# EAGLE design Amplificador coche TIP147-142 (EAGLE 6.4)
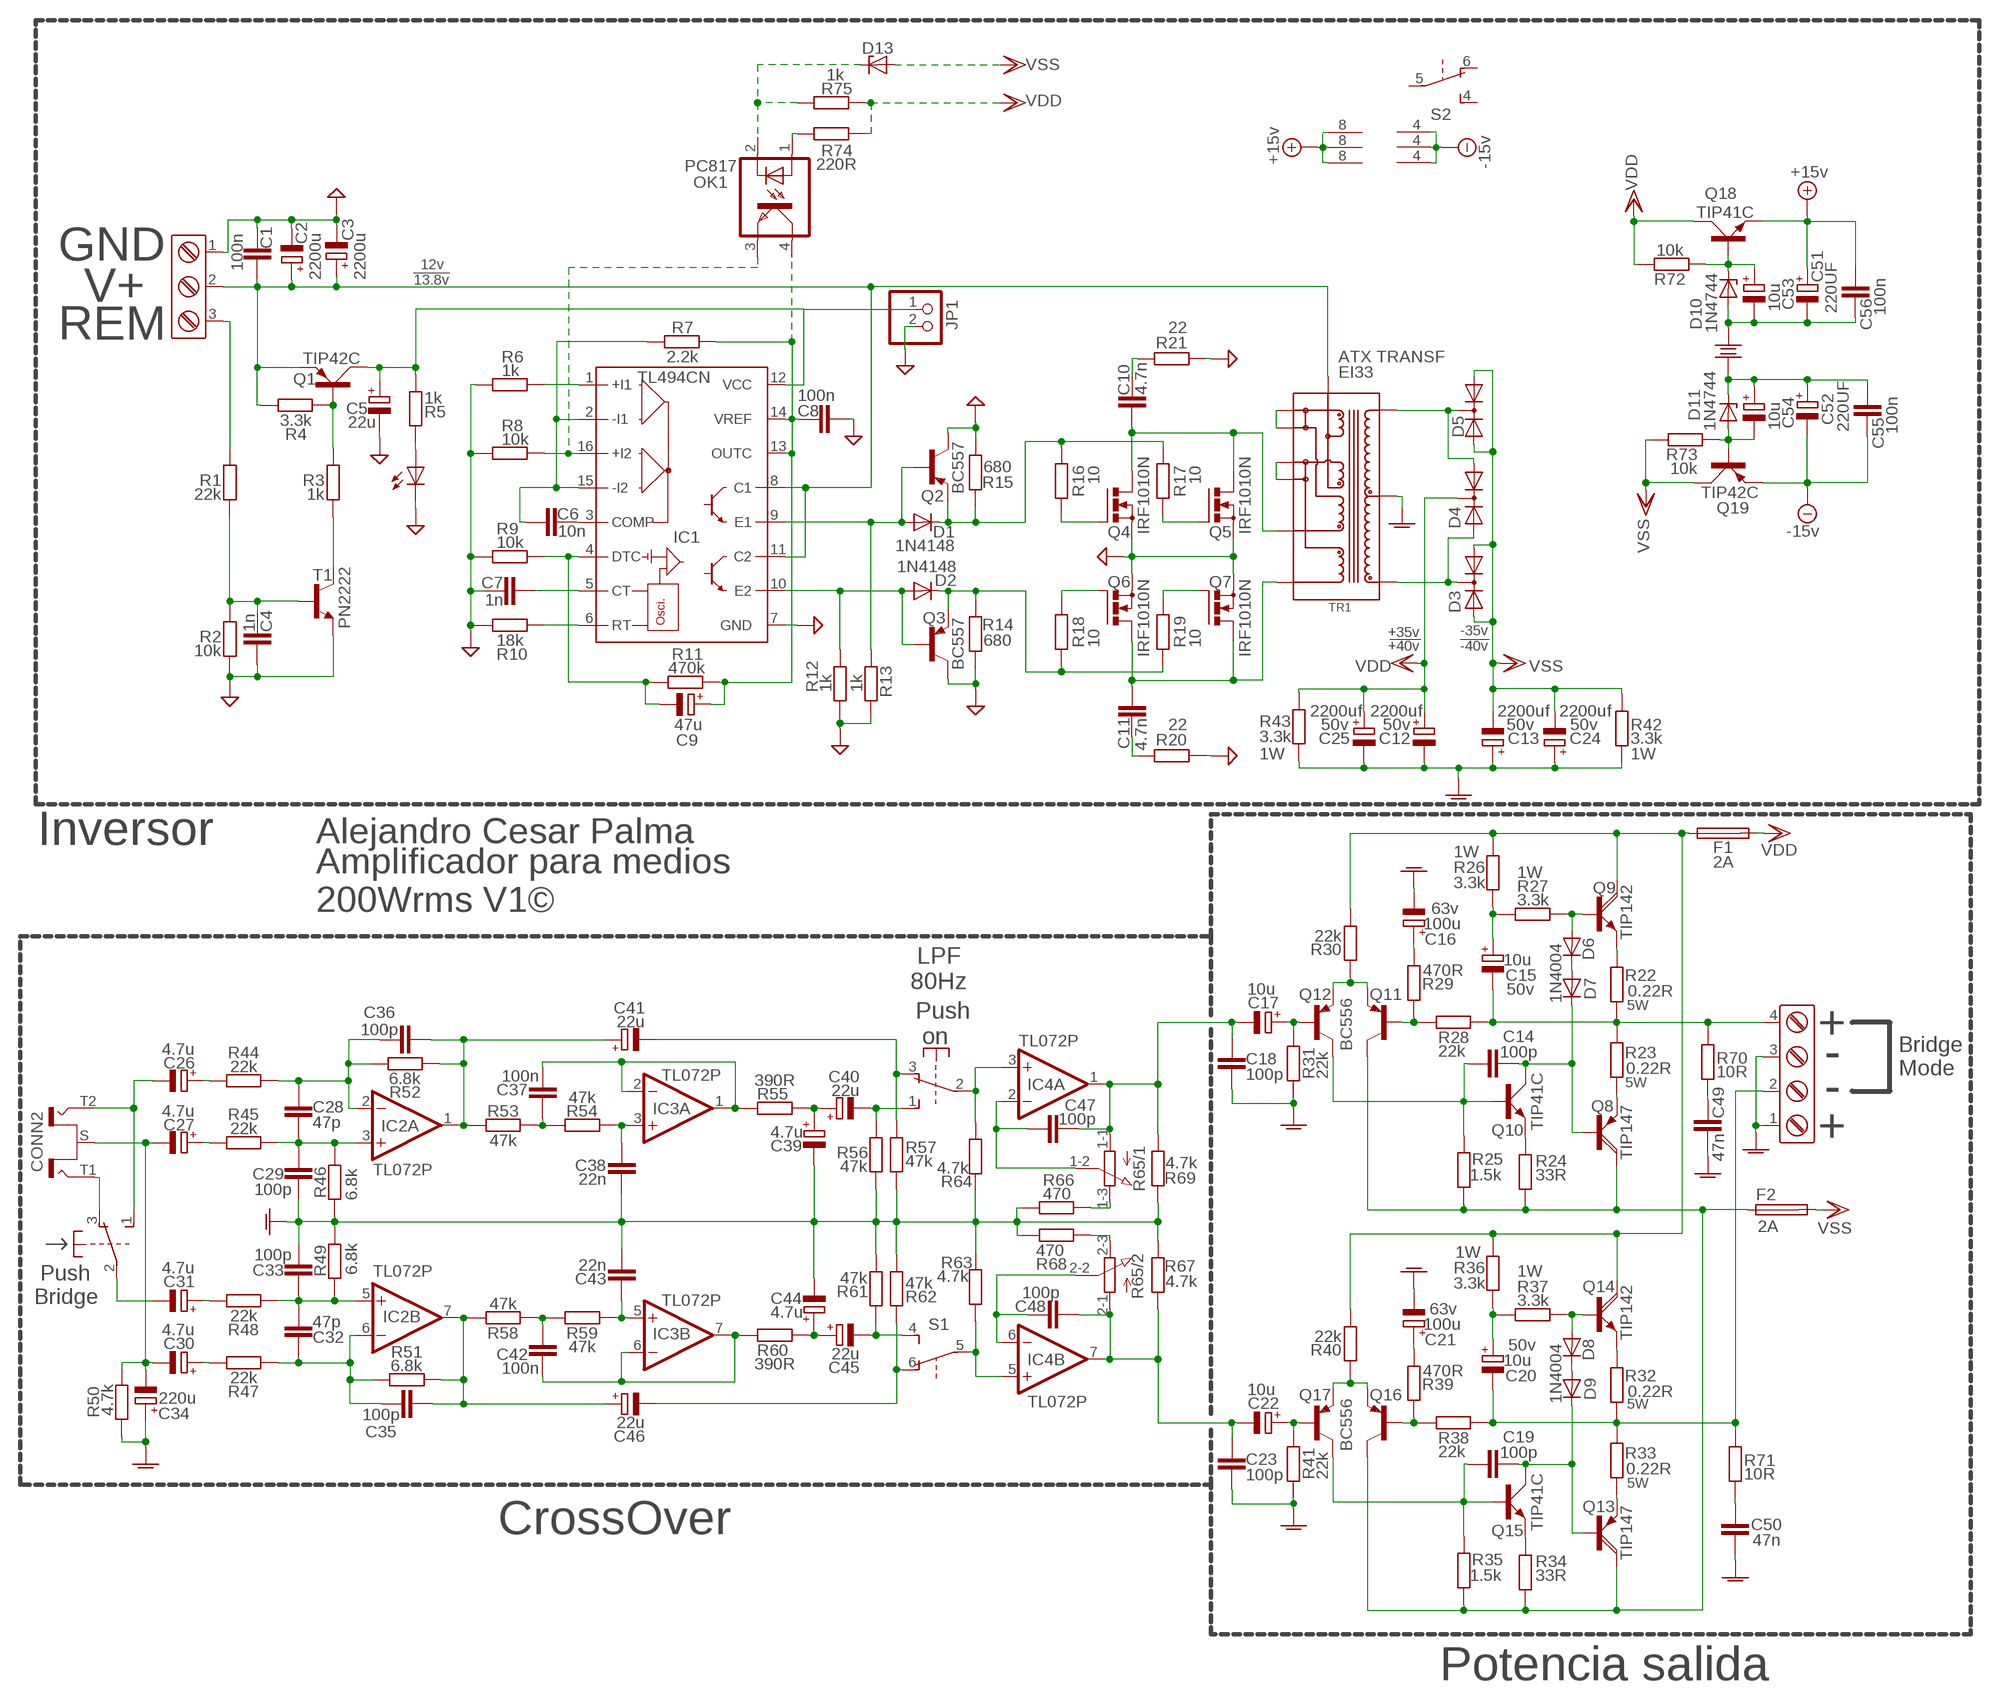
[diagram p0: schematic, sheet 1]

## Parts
C1  100n  C-EU050-024X044  [C050-024X044]
C2  2200u  CPOL-EUE5-13  [E5-13]
C3  2200u  CPOL-EUE5-13  [E5-13]
C4  1n  C-EU050-024X044  [C050-024X044]
C5  22u  CPOL-EUE2.5-5  [E2,5-5]
C6  10n  C-EU050-024X044  [C050-024X044]
C7  1n  C-EU050-024X044  [C050-024X044]
C8  100n  C-EU050-024X044  [C050-024X044]
C9  47u  CPOL-EUE2.5-5  [E2,5-5]
C10  4.7n  C-EU050-024X044  [C050-024X044]
C11  4.7n  C-EU050-024X044  [C050-024X044]
C12  2200uf  CPOL-EUE7.5-18  [E7,5-18]
C13  2200uf  CPOL-EUE7.5-18  [E7,5-18]
C14  100p  C-EU050-024X044  [C050-024X044]
C15  10u  CPOL-EUE2.5-5  [E2,5-5]
C16  100u  CPOL-EUE3.5-8  [E3,5-8]
C17  10u  CPOL-EUE2.5-5  [E2,5-5]
C18  100p  C-EU050-024X044  [C050-024X044]
C19  100p  C-EU050-024X044  [C050-024X044]
C20  10u  CPOL-EUE2.5-5  [E2,5-5]
C21  100u  CPOL-EUE3.5-8  [E3,5-8]
C22  10u  CPOL-EUE2.5-5  [E2,5-5]
C23  100p  C-EU050-024X044  [C050-024X044]
C24  2200uf  CPOL-EUE7.5-18  [E7,5-18]
C25  2200uf  CPOL-EUE7.5-18  [E7,5-18]
C26  4.7u  CPOL-EUE2.5-5  [E2,5-5]
C27  4.7u  CPOL-EUE2.5-5  [E2,5-5]
C28  47p  C-EU050-024X044  [C050-024X044]
C29  100p  C-EU050-024X044  [C050-024X044]
C30  4.7u  CPOL-EUE2.5-5  [E2,5-5]
C31  4.7u  CPOL-EUE2.5-5  [E2,5-5]
C32  47p  C-EU050-024X044  [C050-024X044]
C33  100p  C-EU050-024X044  [C050-024X044]
C34  220u  CPOL-EUE3.5-8  [E3,5-8]
C35  100p  C-EU050-024X044  [C050-024X044]
C36  100p  C-EU050-024X044  [C050-024X044]
C37  100n  C-EU050-024X044  [C050-024X044]
C38  22n  C-EU050-024X044  [C050-024X044]
C39  4.7u  CPOL-EUE2.5-5  [E2,5-5]
C40  22u  CPOL-EUE2.5-5  [E2,5-5]
C41  22u  CPOL-EUE2.5-5  [E2,5-5]
C42  100n  C-EU050-024X044  [C050-024X044]
C43  22n  C-EU050-024X044  [C050-024X044]
C44  4.7u  CPOL-EUE2.5-5  [E2,5-5]
C45  22u  CPOL-EUE2.5-5  [E2,5-5]
C46  22u  CPOL-EUE2.5-5  [E2,5-5]
C47  100p  C-EU050-024X044  [C050-024X044]
C48  100p  C-EU050-024X044  [C050-024X044]
C49  47n  C-EU050-024X044  [C050-024X044]
C50  47n  C-EU050-024X044  [C050-024X044]
C51  220UF  CPOL-EUE5-10.5  [E5-10,5]
C52  220UF  CPOL-EUE5-10.5  [E5-10,5]
C53  10u  CPOL-EUE2.5-5  [E2,5-5]
C54  10u  CPOL-EUE2.5-5  [E2,5-5]
C55  100n  C-EU050-024X044  [C050-024X044]
C56  100n  C-EU050-024X044  [C050-024X044]
CON1  CONECTOR_DEGSON_4_PIN  [CONN_DEGSON_4_PIN]
CONN1  CONECTOR_DEGSON_3_PIN  [CONN_DEGSON_3_PIN]
CONN2  RCA-2-VERT-V2  [RCA-2-VERT_V2]
D1  1N4148  1N4148DO35-7  [DO35-7]
D2  1N4148  1N4148DO35-7  [DO35-7]
D3  FEP16AT  [TO220ABS]
D4  FEP16AT  [TO220ABS]
D5  FEP16AT  [TO220ABS]
D6  1N4004  [DO41-10]
D7  1N4004  [DO41-10]
D8  1N4004  [DO41-10]
D9  1N4004  [DO41-10]
D10  1N4744  ZENER-DIODEDO34-7  [DO34Z7]
D11  1N4744  ZENER-DIODEDO34-7  [DO34Z7]
D13  ZENER-DIODEDO34-7  [DO34Z7]
F1  FUSESHK20L  [SHK20L]
F2  FUSESHK20L  [SHK20L]
IC1  TL494CN  [DIL16]
IC2  TL072P  [DIL08]
IC3  TL072P  [DIL08]
IC4  TL072P  [DIL08]
JP1  PINHD-1X2  [1X02]
LED1  LED3MM  [LED3MM]
OK1  PC817  [DIL04]
Q1  TIP42C  [TO220AV]
Q2  BC557  [TO92-EBC]
Q3  BC557  [TO92-EBC]
Q4  IRF1010N  BUZ11BV  [TO220BV]
Q5  IRF1010N  BUZ11BV  [TO220BV]
Q6  IRF1010N  BUZ11BV  [TO220BV]
Q7  IRF1010N  BUZ11BV  [TO220BV]
Q8  TIP147  [TO247BV]
Q9  TIP142  [TO247BV]
Q10  TIP41C  [TO220AV]
Q11  BC556  [TO92-EBC]
Q12  BC556  [TO92-EBC]
Q13  TIP147  [TO247BV]
Q14  TIP142  [TO247BV]
Q15  TIP41C  [TO220AV]
Q16  BC556  [TO92-EBC]
Q17  BC556  [TO92-EBC]
Q18  TIP41C  [TO220AV]
Q19  TIP42C  [TO220AV]
R1  22k  R-EU_0207/7  [0207/7]
R2  10k  R-EU_0207/7  [0207/7]
R3  1k  R-EU_0207/7  [0207/7]
R4  3.3k  R-EU_0207/7  [0207/7]
R5  1k  R-EU_0207/7  [0207/7]
R6  1k  R-EU_0207/7  [0207/7]
R7  2.2k  R-EU_0207/7  [0207/7]
R8  10k  R-EU_0207/7  [0207/7]
R9  10k  R-EU_0207/7  [0207/7]
R10  18k  R-EU_0207/7  [0207/7]
R11  470k  R-EU_0207/7  [0207/7]
R12  1k  R-EU_0207/7  [0207/7]
R13  1k  R-EU_0207/7  [0207/7]
R14  680  R-EU_0207/7  [0207/7]
R15  680  R-EU_0207/7  [0207/7]
R16  10  R-EU_0207/7  [0207/7]
R17  10  R-EU_0207/7  [0207/7]
R18  10  R-EU_0207/7  [0207/7]
R19  10  R-EU_0207/7  [0207/7]
R20  22  R-EU_0207/7  [0207/7]
R21  22  R-EU_0207/7  [0207/7]
R22  0.22R  R-EU_VTA53  [VTA53]
R23  0.22R  R-EU_VTA53  [VTA53]
R24  33R  R-EU_0207/7  [0207/7]
R25  1.5k  R-EU_0207/7  [0207/7]
R26  3.3k  R-EU_0411/12  [0411/12]
R27  3.3k  R-EU_0411/12  [0411/12]
R28  22k  R-EU_0207/7  [0207/7]
R29  470R  R-EU_0207/7  [0207/7]
R30  22k  R-EU_0207/7  [0207/7]
R31  22k  R-EU_0207/7  [0207/7]
R32  0.22R  R-EU_VTA53  [VTA53]
R33  0.22R  R-EU_VTA53  [VTA53]
R34  33R  R-EU_0207/7  [0207/7]
R35  1.5k  R-EU_0207/7  [0207/7]
R36  3.3k  R-EU_0411/12  [0411/12]
R37  3.3k  R-EU_0411/12  [0411/12]
R38  22k  R-EU_0207/7  [0207/7]
R39  470R  R-EU_0207/7  [0207/7]
R40  22k  R-EU_0207/7  [0207/7]
R41  22k  R-EU_0207/7  [0207/7]
R42  3.3k  R-EU_0411/12  [0411/12]
R43  3.3k  R-EU_0411/12  [0411/12]
R44  22k  R-EU_0207/7  [0207/7]
R45  22k  R-EU_0207/7  [0207/7]
R46  6.8k  R-EU_0207/7  [0207/7]
R47  22k  R-EU_0207/7  [0207/7]
R48  22k  R-EU_0207/7  [0207/7]
R49  6.8k  R-EU_0207/7  [0207/7]
R50  4.7k  R-EU_0207/7  [0207/7]
R51  6.8k  R-EU_0207/7  [0207/7]
R52  6.8k  R-EU_0207/7  [0207/7]
R53  47k  R-EU_0207/7  [0207/7]
R54  47k  R-EU_0207/7  [0207/7]
R55  390R  R-EU_0207/7  [0207/7]
R56  47k  R-EU_0207/7  [0207/7]
R57  47k  R-EU_0207/7  [0207/7]
R58  47k  R-EU_0207/7  [0207/7]
R59  47k  R-EU_0207/7  [0207/7]
R60  390R  R-EU_0207/7  [0207/7]
R61  47k  R-EU_0207/7  [0207/7]
R62  47k  R-EU_0207/7  [0207/7]
R63  4.7k  R-EU_0207/7  [0207/7]
R64  4.7k  R-EU_0207/7  [0207/7]
R65  3RP/1610G  [3RP/1610G]
R66  470  R-EU_0207/7  [0207/7]
R67  4.7k  R-EU_0207/7  [0207/7]
R68  470  R-EU_0207/7  [0207/7]
R69  4.7k  R-EU_0207/7  [0207/7]
R70  10R  R-EU_0411/12  [0411/12]
R71  10R  R-EU_0411/12  [0411/12]
R72  10k  R-EU_0207/7  [0207/7]
R73  10k  R-EU_0207/7  [0207/7]
R74  220R  R-EU_0207/7  [0207/7]
R75  1k  R-EU_0207/7  [0207/7]
S1  9077-2  [9077-2]
S2  9077-2  [9077-2]
T1  PN2222  2N2222-NPN-TO92-EBC  [TO92-EBC]
TR1  ATX1  [ATX/300W]

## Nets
+14V: C51.+ C56.2 IC2.8(P:V+) IC3.8(P:V+) IC4.8(P:V+) Q18.E ; supply symbol labelled +15v
-14V: C52.- C55.1 IC2.4(P:V-) IC3.4(P:V-) IC4.4(P:V-) Q19.E ; supply symbol labelled -15v
GND: C1.1 C2.- C3.- C4.2 C5.- C7.1 C8.2 CONN1.1 IC1.7(GND) JP1.2 LED1.K(C) Q2.C Q3.C Q4.S Q5.S Q6.S Q7.S R2.1 R6.2 R8.2 R9.2 R10.2 R12.2 R13.2 R14.2 R15.2 R20.2 R21.2 T1.E
GNDA: C12.- C13.+ C16.- C18.1 C21.- C23.1 C24.+ C25.- C29.1 C33.1 C34.+ C38.2 C39.- C43.2 C44.- C49.1 C50.1 C51.- C52.+ C53.- C54.+ C55.2 C56.1 CON1.1 CON1.3 D10.A D11.C R31.1 R41.1 R42.2 R43.2 R46.1 R49.1 R50.2 R56.2 R57.2 R61.2 R62.2 R63.1 R64.1 R66.2 R67.1 R68.2 R69.1 TR1.9
N$1: C1.2 C2.+ C3.+ CONN1.2 IC1.8(C1) IC1.11(C2) Q1.E R4.2 TR1.7
N$2: C26.+ R44.1
N$3: CONN1.3 R1.2
N$4: C4.1 R1.1 R2.2 T1.B
N$5: R3.1 T1.C
N$6: Q1.B R3.2 R4.1
N$7: C5.+ IC1.12(VCC) JP1.1 Q1.C R5.1
N$8: LED1.A R5.2
N$9: OK1.1(A) R74.1
N$10: C6.2 IC1.3(COMP)
N$11: C6.1 IC1.2(-I1) IC1.15(-I2) R7.2
N$12: C8.1 C9.+ IC1.13(OUTC) IC1.14(VREF) OK1.4(COL) R7.1 R11.1
N$13: IC1.16(+I2) OK1.3(EMIT) R8.1
N$14: Q4.G R16.1
N$15: C9.- IC1.4(DTC) R9.1 R11.2
N$16: C7.2 IC1.5(CT)
N$17: IC1.6(RT) R10.1
N$18: Q5.G R17.1
N$19: C11.2 R20.1
N$20: D2.A IC1.10(E2) Q3.B R12.1
N$21: D1.A IC1.9(E1) Q2.B R13.1
N$22: D1.C Q2.E R15.1 R16.2 R17.2
N$23: Q6.G R18.1
N$24: D2.C Q3.E R14.1 R18.2 R19.2
N$25: Q7.G R19.1
N$26: C10.1 Q4.D Q5.D TR1.2
N$27: C11.1 Q6.D Q7.D TR1.1
N$28: C10.2 R21.1
N$29: IC1.1(+I1) R6.1
N$30: TR1.3 TR1.4
N$31: TR1.5 TR1.6
N$32: C27.+ R45.1
N$33: D3.C D4.A2 TR1.10
N$34: D4.A1 D5.C TR1.8
N$35: Q9.S(E) R22.2
N$36: C15.- CON1.4 R22.1 R23.2 R28.2 R70.1
N$37: Q8.S(E) R23.1
N$38: D6.A Q9.G(B) R27.2
N$39: D6.C D7.A
N$40: C14.2 D7.C Q8.G(B) Q10.C
N$41: Q10.E R24.1
N$42: C28.2 C36.1 IC2.2(A:-IN) R44.2 R52.1
N$43: C15.+ R26.2 R27.1
N$44: C14.1 Q10.B Q12.C R25.1
N$45: Q11.B R28.1 R29.1
N$46: C28.1 C29.2 IC2.3(A:+IN) R45.2 R46.2
N$47: Q11.E Q12.E R30.1
N$48: C16.+ R29.2
N$49: C17.+ Q12.B R31.2
N$50: CONN2.T1 S2.3(1:O)
N$51: Q14.S(E) R32.2
N$52: C20.- CON1.2 R32.1 R33.2 R38.2 R71.1
N$53: Q13.S(E) R33.1
N$54: D8.A Q14.G(B) R37.2
N$55: D8.C D9.A
N$56: C19.2 D9.C Q13.G(B) Q15.C
N$57: Q15.E R34.1
N$58: C27.- C30.- C34.- CONN2.S R50.1
N$59: C19.1 Q15.B Q17.C R35.1
N$60: C20.+ R36.2 R37.1
N$61: C30.+ R47.1
N$62: Q16.B R38.1 R39.1
N$63: Q16.E Q17.E R40.1
N$64: C21.+ R39.2
N$65: C22.+ Q17.B R41.2
N$66: C49.2 R70.2
N$67: C31.+ R48.1
N$68: C32.2 C35.1 IC2.6(B:-IN) R47.2 R51.1
N$69: C32.1 C33.2 IC2.5(B:+IN) R48.2 R49.2
N$70: C35.2 C46.+ IC2.7(B:OUT) R51.2 R58.1
N$71: C26.- CONN2.T2 S2.1(1:S)
N$72: C31.- S2.2(1:P)
N$73: C37.1 R53.2 R54.1
N$74: C36.2 C41.+ IC2.1(A:OUT) R52.2 R53.1
N$75: C38.1 IC3.3(A:+IN) R54.2
N$76: C37.2 IC3.1(A:OUT) IC3.2(A:-IN) R55.2
N$77: C39.+ C40.+ R55.1
N$78: C40.- R56.1 S1.1(1:S)
N$79: C41.- R57.1 S1.3(1:O)
N$80: IC4.5(B:+IN) R63.2 S1.5(2:P)
N$81: C42.1 R58.2 R59.1
N$82: C43.1 IC3.5(B:+IN) R59.2
N$83: C42.2 IC3.6(B:-IN) IC3.7(B:OUT) R60.2
N$84: C44.+ C45.+ R60.1
N$85: C45.- R61.1 S1.4(2:S)
N$86: C46.- R62.1 S1.6(2:O)
N$87: IC4.3(A:+IN) R64.2 S1.2(1:P)
N$88: C47.1 IC4.2(A:-IN) R65.1-2(/1:S)
N$89: C17.- C18.2 C47.2 IC4.1(A:OUT) R65.1-1(/1:A) R69.2
N$90: R65.1-3(/1:E) R66.1
N$91: D13.C OK1.2(C) R75.2
N$92: C48.1 IC4.6(B:-IN) R65.2-2(/2:S)
N$93: C22.- C23.2 C48.2 IC4.7(B:OUT) R65.2-1(/2:A) R67.2
N$94: R65.2-3(/2:E) R68.1
N$95: C50.2 R71.2
N$99: F1.1A Q9.D(C) Q14.D(C) R26.1 R30.2 R36.1 R40.2
N$101: C53.+ D10.C Q18.B R72.1
N$102: C54.- D11.A Q19.B R73.1
N$104: F2.1A Q8.D(C) Q11.C Q13.D(C) Q16.C R24.2 R25.2 R34.2 R35.2
VDD: C12.+ C25.+ D4.C F1.2A Q18.C R43.1 R72.2 R74.2 R75.1
VSS: C13.- C24.- D3.A1 D3.A2 D5.A1 D5.A2 D13.A F2.2A Q19.C R42.1 R73.2
Unconnected: S2.4(2:S) S2.5(2:P) S2.6(2:O)

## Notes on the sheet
- GND
- 12v
- 13.8v
- V+
- REM
- ATX TRANSF
- EI33
- +35v | -35v
- +40v | -40v
- 50v | 50v | 50v | 50v
- 1W | 1W
- Inversor | Alejandro Cesar Palma
- 1W
- 2A
- 1W
- Amplificador para medios
  200Wrms V1©
- 63v
- LPF
  80Hz
- 50v
- 5W
- +
- Push
   on
- -
- Bridge
  Mode
- 5W
- -
- +
- 2A
- 1W
- 1W
- Push
  Bridge
- 63v
- 50v
- 5W
- 5W
- CrossOver
- Potencia salida

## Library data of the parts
C1 C4 C6-C8 C10 C11 C14 C18 C19 C23 C28 C29 C32 C33 C35-C38 C42 C43 C47-C50 C55 C56 = rcl:C-EU: CAPACITOR, European symbol
C2 C3 C5 C9 C12 C13 C15-C17 C20-C22 C24-C27 C30 C31 C34 C39-C41 C44-C46 C51-C54 = rcl:CPOL-EU: POLARIZED CAPACITOR, European symbol
CON1 = conector_car_audio:CONECTOR_DEGSON_4_PIN
CONN1 = conector_car_audio:CONECTOR_DEGSON_3_PIN
CONN2 = con-amphenol:RCA-2-VERT-V2
D1 D2 = diode:1N4148: DIODE
D3-D5 = diode:FEP16AT: DIODE dual ultra-fast recovery rectifier, common cathode
D6-D9 = diode-1:1N4004: DIODE
D10 D11 D13 = diode:ZENER-DIODE: Z-Diode
F1 F2 = fuse:FUSE: Fuse; OC_FARNELL: unknown; OC_NEWARK: unknown
IC1 = linear:TL494*: SWITCHMODE Pulse Width Modulation Control Circuit NCV494B http://onsemi.com tl494-d.pdf
IC2-IC4 = linear:TL072: OP AMP
JP1 = pinhead:PINHD-1X2: PIN HEADER
LED1 = led:LED: LED
OK1 = optocoupler:PC817: SHARP OPTO COUPLER; MPN: PC817X4J000F; OC_FARNELL: 9707727; OC_NEWARK: 97K7059
Q1 Q19 = transistor-power:TIP42C: PNP TRANSISTOR
Q2 Q3 = transistor-pnp:BC557*: PNP Transistror
Q4-Q7 = transistor-power:BUZ11: N-CHANNEL MOS FET
Q8 Q13 = transistor-power:TIP147: PNP DARLINGTON TRANSISTOR
Q9 Q14 = transistor-power:TIP142: NPN DARLINGTON TRANSISTOR
Q10 Q15 Q18 = transistor-power:TIP41C: NPN TRANSISTOR
Q11 Q12 Q16 Q17 = transistor-pnp:BC556*: PNP Transistror
R1-R64 R66-R75 = rcl:R-EU_: RESISTOR, European symbol
R65 = pot:3RP/1610G: 16mm Potentiometer two level Source: http://www.alphapotentiometers.net/html/16mm_pot_2.html
S1 S2 = switch-misc:9077-2: MARQUARDT SWITCH 9077.0200 Distributor: Buerklin
T1 = transistor-neu-to92:*-NPN-: NPN Transistror
TR1 = ATX:ATX1

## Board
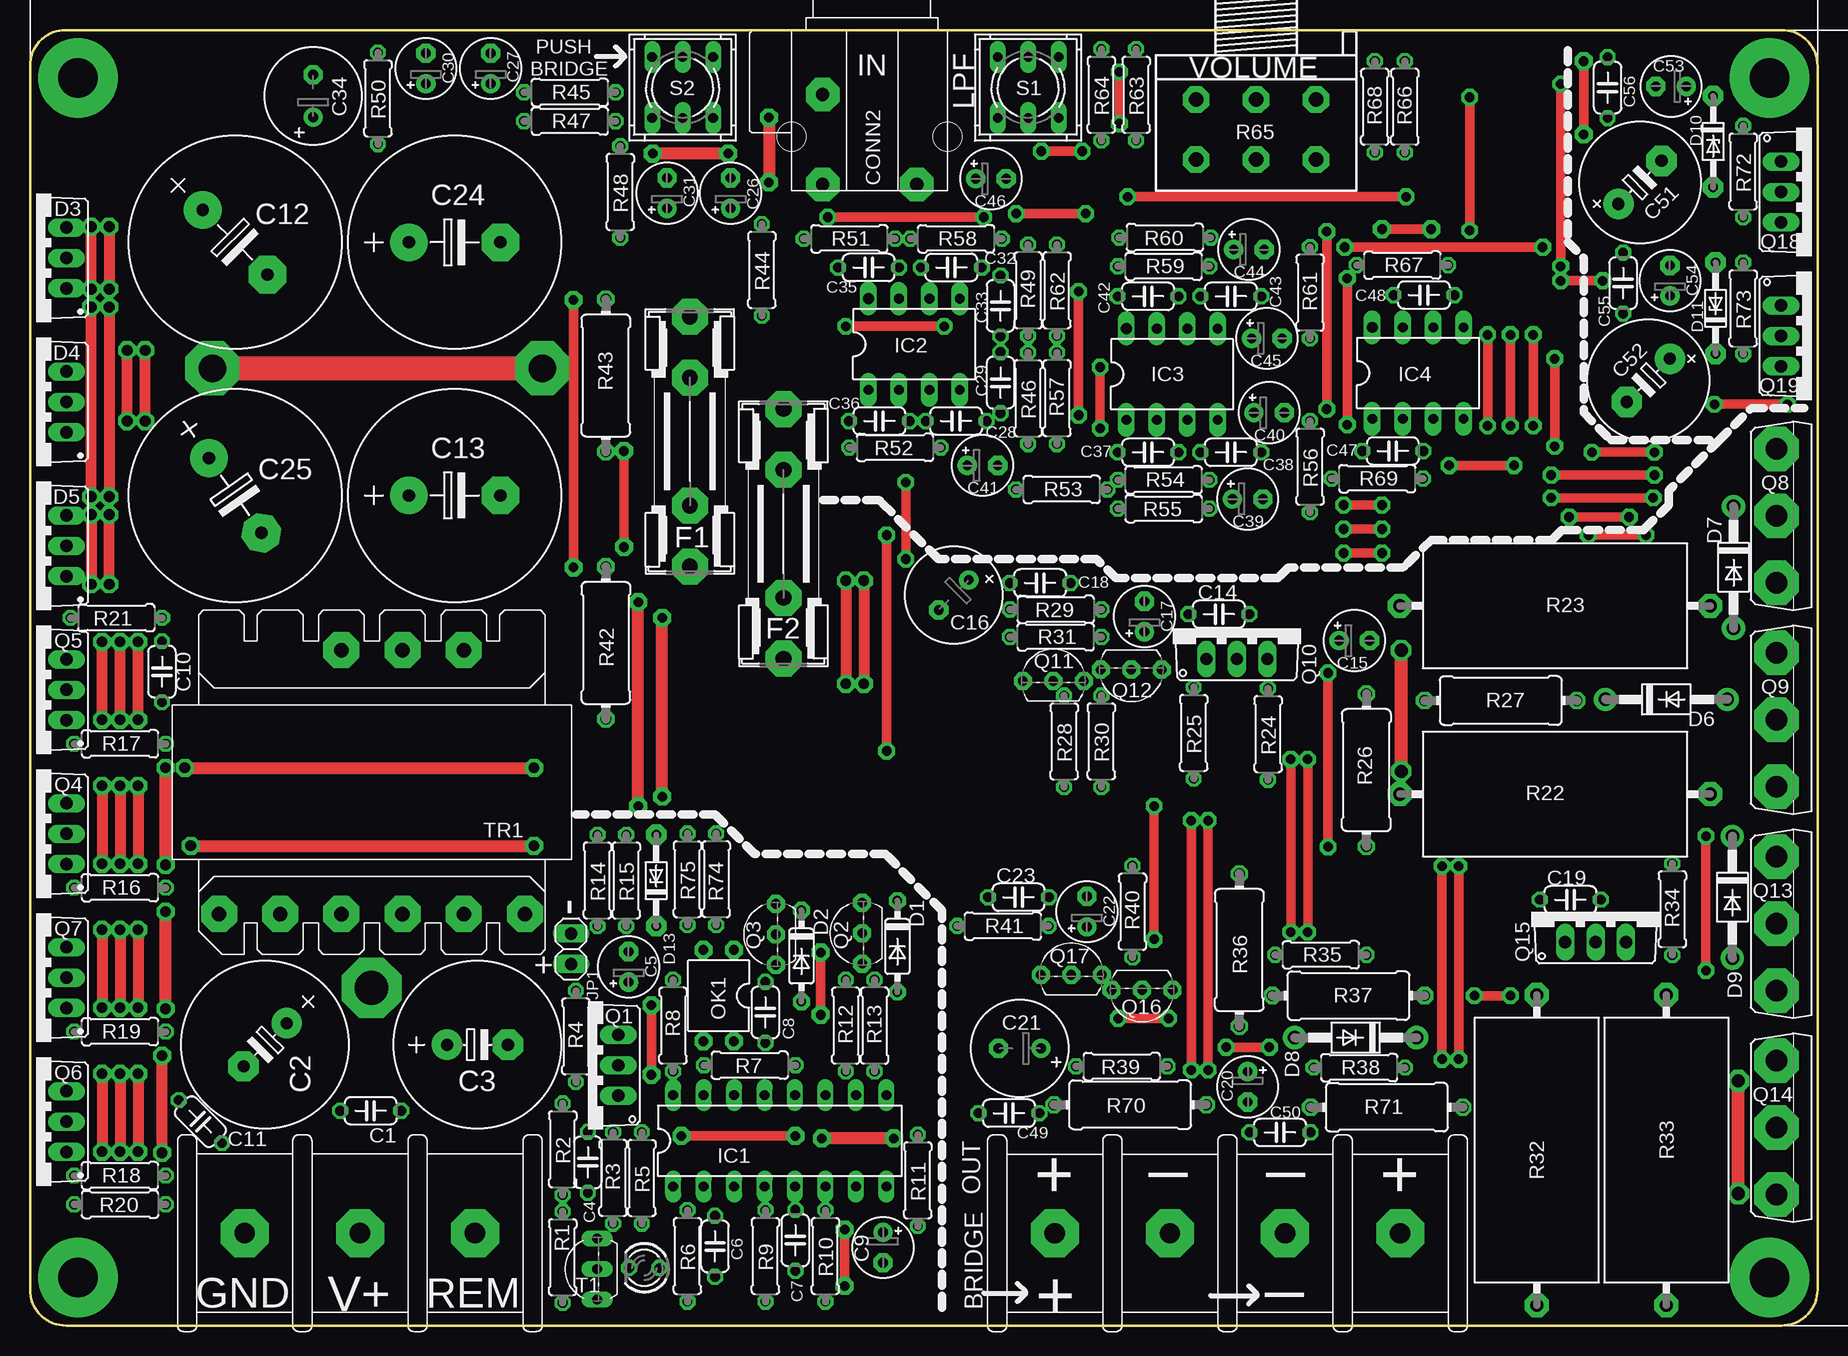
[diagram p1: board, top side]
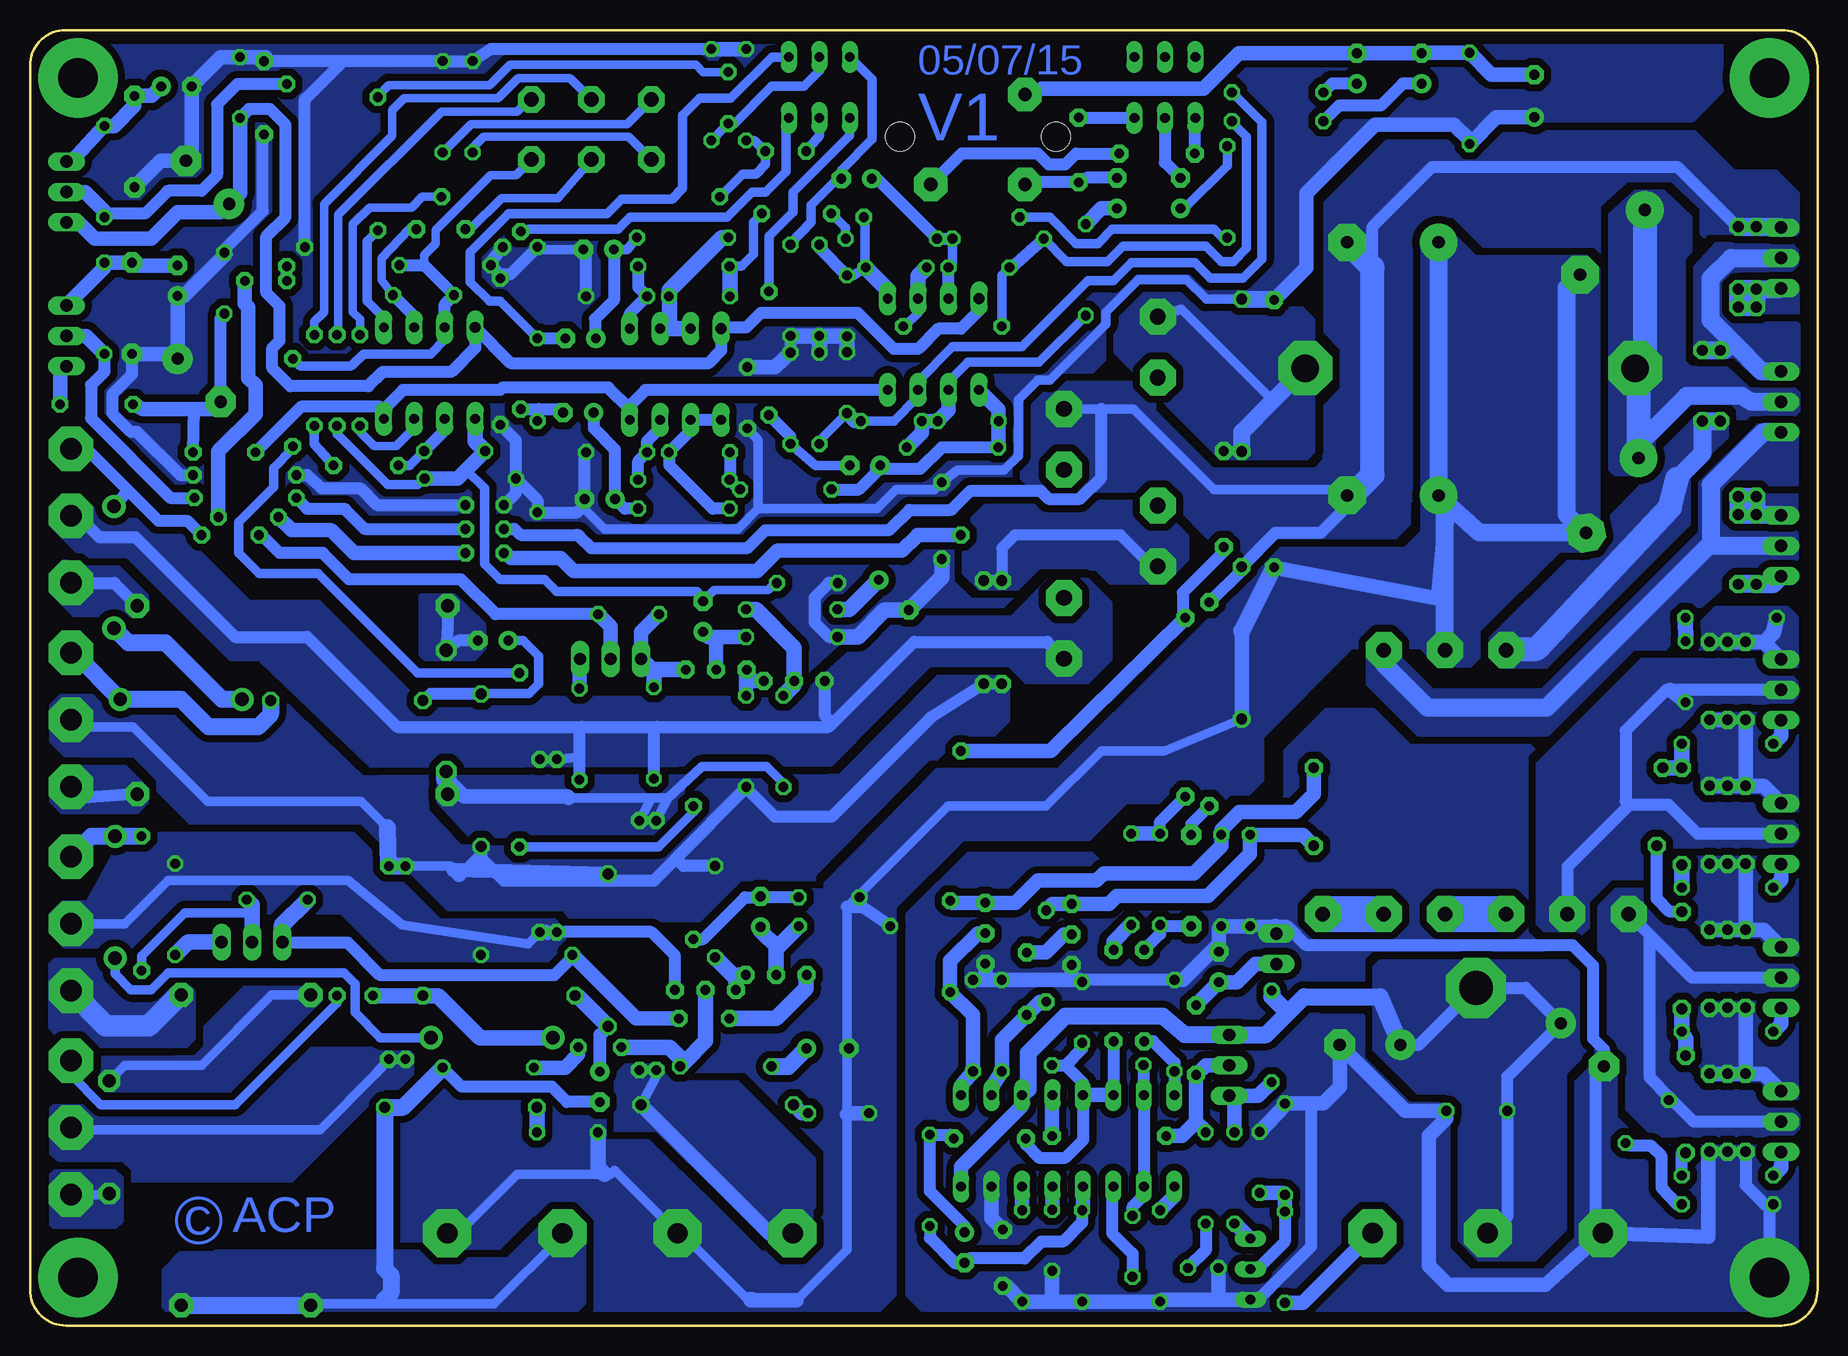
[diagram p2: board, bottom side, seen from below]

Size 149 x 108 mm. Coordinates in mm from the lower left corner, seen from the top.
Outline: 3,0 146,0 arc90 149,3 149,105 arc90 146,108 3,108 arc90 0,105 0,3 arc90 3,0
Copper layers (1*16): Top 0.035mm / dielectric 1.5mm / Bottom 0.035mm
Design rules "default": minimum track width 10mil, minimum drill 24mil, track to track 8mil, track to pad 8mil, pad to pad 8mil, via to via 8mil, smd to smd 8mil, copper to edge 40mil, drill to drill 8mil, minimum pad ring 10mil, minimum via ring 8mil, stop-mask expansion 4mil, vias tented up to drill 0mil, thermal gap 10mil

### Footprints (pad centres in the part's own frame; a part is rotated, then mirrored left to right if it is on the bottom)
C050-024X044 = drill 0.813 octagon: 1 -2.54,0; 2 2.54,0
E5-13 = drill 1.016 pad 2.54: + -2.54,0 | drill 1.016 pad 2.54 octagon: - 2.54,0
E2,5-5 = drill 0.813 pad 1.6: + -1.27,0 | drill 0.813 pad 1.6 octagon: - 1.27,0
E7,5-18 = drill 1.016 pad 3.15: + -3.81,0 | drill 1.016 pad 3.15 octagon: - 3.81,0
E3,5-8 = drill 0.813 pad 1.6: + -1.778,0 | drill 0.813 pad 1.6 octagon: - 1.778,0
E5-10,5 = drill 1.016 pad 2.54: + -2.54,0 | drill 1.016 pad 2.54 octagon: - 2.54,0
CONN_DEGSON_4_PIN = drill 1.7 pad 4 octagon: 1 -6.12,-0.59; 2 3.48,-0.59; 3 13.08,-0.59; 4 22.68,-0.59
CONN_DEGSON_3_PIN = drill 1.7 pad 4 octagon: 1 -10.7,6.8; 2 -1.1,6.8; 3 8.5,6.8
RCA-2-VERT_V2 = drill 1.1 pad 2.8 octagon: S -3.33,5.22; T1 4.52,-2.28; T2 -3.33,-2.28 | hole 2.4: -5.93,1.72; 7.07,1.72
DO35-7 = drill 0.813 pad 1.4 octagon: A 3.81,0; C -3.81,0
TO220ABS = drill 1.016 long: A1 -2.54,-2.54; A2 2.54,-2.54; C 0,-2.54
DO41-10 = drill 1.118 pad 1.93: A 5.08,0; C -5.08,0
DO34Z7 = drill 0.813 pad 1.7 octagon: A 3.81,0; C -3.81,0
SHK20L = drill 1.321 pad 3 octagon: 1A -10.414,0; 1B -5.334,0; 2A 10.414,0; 2B 5.334,0
DIL16 = drill 0.813 long: 1 -8.89,-3.81; 2 -6.35,-3.81; 3 -3.81,-3.81; 4 -1.27,-3.81; 5 1.27,-3.81; 6 3.81,-3.81; 7 6.35,-3.81; 8 8.89,-3.81; 9 8.89,3.81; 10 6.35,3.81; 11 3.81,3.81; 12 1.27,3.81; 13 -1.27,3.81; 14 -3.81,3.81; 15 -6.35,3.81; 16 -8.89,3.81
DIL08 = drill 0.813 pad 1.4 long: 1 -3.81,-3.81; 2 -1.27,-3.81; 3 1.27,-3.81; 4 3.81,-3.81; 5 3.81,3.81; 6 1.27,3.81; 7 -1.27,3.81 | drill 0.9 pad 1.4 long: 8 -3.81,3.81
1X02 = drill 1.016 long: 1 -1.27,0; 2 1.27,0
LED3MM = drill 0.813 octagon: A -1.27,0; K 1.27,0
DIL04 = drill 0.813 pad 1.5 octagon: 1 -1.27,-3.81; 2 1.27,-3.81; 3 1.27,3.81; 4 -1.27,3.81
TO220AV = drill 1.016 long: B -2.54,-2.54; C 0,-2.54; E 2.54,-2.54
TO92-EBC = drill 0.813 pad 1.5 octagon: B 0,-1.27; C -2.54,-1.27; E 2.54,-1.27
TO220BV = drill 1.016 long: D 0,-2.54; G -2.54,-2.54; S 2.54,-2.54
TO247BV = drill 1.8 pad 3.7 octagon: D 0,-2.921; G -5.588,-2.921; S 5.588,-2.921
0207/7 = drill 0.813 octagon: 1 -3.81,0; 2 3.81,0
VTA53 = drill 1.1 pad 2 octagon: 1 -11.815,0; 2 14.065,0
0411/12 = drill 0.914 octagon: 1 -6.35,0; 2 6.35,0
3RP/1610G = drill 1.2 pad 2.2 octagon: 1-1 -5,0; 1-2 0,0; 1-3 5,0; 2-1 -5,5; 2-2 0,5; 2-3 5,5
9077-2 = drill 0.813 long: 1 -2.54,2.54; 2 0,2.54; 3 2.54,2.54; 4 -2.54,-2.54; 5 0,-2.54; 6 2.54,-2.54
TO92-EBC' = drill 0.813 long: B 0,-1.27; C 2.54,-1.27; E -2.54,-1.27
ATX/300W = drill 1.2 pad 3 octagon: 1 -10.9,13.65; 2 -10.9,8.55; 3 -10.9,3.45; 4 -10.9,-1.65; 5 -10.9,-6.75; 6 -10.9,-11.85; 8 11.1,-6.75; 9 11.1,-1.65; 10 11.1,3.45 | drill 2.8 pad 5 octagon: 7 -17.05,0.94

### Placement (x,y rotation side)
C1  28.4,17.9 180 top
C2  19.6,23.4 225 top
C3  37.3,23.4 0 top
C4  46.5,13.6 90 top
C5  49.9,29.9 90 top
C6  57.1,6.6 270 top
C7  63.8,7.1 90 top
C8  61.3,26.1 90 top
C9  71.1,6.5 270 top
C10  11,54.5 90 top
C11  14.2,17 315 top
C12  17.1,90.3 315 top
C13  35.4,69.2 0 top
C14  99.1,59.3 0 top
C15  110.4,57.1 0 top
C16  77,60.9 225 top
C17  92.9,59.1 90 top
C18  84.2,61.9 0 top
C19  128.4,35.5 0 top
C20  101.5,19.9 270 top
C21  82.5,23.1 180 top
C22  88.1,34.5 90 top
C23  82.4,35.7 0 top
C24  35.4,90.3 0 top
C25  17.1,69.2 305 top
C26  58.4,94.4 90 top
C27  38.4,104.8 90 top
C28  77.2,75.4 180 top
C29  80.9,78.6 270 top
C30  33,104.8 90 top
C31  53.1,94.4 90 top
C32  76.8,88.2 180 top
C33  80.9,85 90 top
C34  23.6,102.5 90 top
C35  69.9,88.2 0 top
C36  70.8,75.4 180 top
C37  93.2,72.8 0 top
C38  100.1,72.8 0 top
C39  101.5,68.9 0 top
C40  103.3,76.1 0 top
C41  79.4,71.7 0 top
C42  93.2,85.8 0 top
C43  100.1,85.8 0 top
C44  101.6,89.7 0 top
C45  103.1,82.3 0 top
C46  80.1,95.6 0 top
C47  113.6,72.9 180 top
C48  116.2,85.9 180 top
C49  81.6,17.7 0 top
C50  104.2,16.1 0 top
C51  134.2,95.3 45 top
C52  134.9,78.8 225 top
C53  136.8,103.3 180 top
C54  136.7,87.1 90 top
C55  132.8,86.9 90 top
C56  131.5,103.2 270 top
CON1  108.1,7.1 180 top
CONN1  28.6,0.9 0 top
CONN2  69.4,97.4 0 top
D1  72.3,31.6 270 top
D2  64.3,30.8 270 top
D3  0.5,89 90 top
D4  0.5,77 90 top
D5  0.5,65 90 top
D6  136.4,52.2 0 top
D7  142,63.2 270 top
D8  110.5,24 180 top
D9  141.9,35.7 270 top
D10  140.3,98.7 270 top
D11  140.5,84.8 90 top
D13  52.2,37.1 90 top
F1  55,73.7 90 top
F2  62.8,66 90 top
IC1  62.5,15.4 0 top
IC2  73.7,81.8 0 top
IC3  95.2,79.3 0 top
IC4  115.7,79.4 0 top
JP1  45.1,31.4 90 top
LED1  51.2,4.8 180 top
OK1  57.4,27.5 180 top
Q1  46.5,21.7 90 top
Q2  68.1,32.7 90 top
Q3  60.9,32.6 90 top
Q4  0.5,41 90 top
Q5  0.5,53 90 top
Q6  0.5,17 90 top
Q7  0.5,29 90 top
Q8  148.5,67.5 270 top
Q9  148.5,50.5 270 top
Q10  100.6,58.1 0 top
Q11  85.3,55 0 top
Q12  91.8,53.4 180 top
Q13  148.5,33.5 270 top
Q14  148.5,16.5 270 top
Q15  130.5,34.5 0 top
Q16  92.7,26.7 180 top
Q17  86.8,30.5 0 top
Q18  148.5,94.5 270 top
Q19  148.5,82.5 270 top
R1  44.4,5.7 270 top
R2  44.4,14.7 270 top
R3  48.6,12.3 90 top
R4  45.5,24.1 90 top
R5  51,12.3 270 top
R6  54.8,5.8 270 top
R7  60,21.7 180 top
R8  53.6,25 90 top
R9  61.3,5.8 270 top
R10  66.3,5.8 270 top
R11  74,12.1 270 top
R12  68,25 90 top
R13  70.4,25 90 top
R14  47.3,37.1 270 top
R15  49.7,37.1 270 top
R16  7.5,36.5 0 top
R17  7.5,48.5 0 top
R18  7.5,12.5 0 top
R19  7.5,24.5 0 top
R20  7.5,10.1 180 top
R21  7.2,59 180 top
R22  126,44.3 0 top
R23  128.25,60 180 top
R24  103.2,49.3 270 top
R25  97,49.4 270 top
R26  111.4,46.3 90 top
R27  122.6,52.1 0 top
R28  86.2,48.7 270 top
R29  85.5,59.7 180 top
R30  89.3,48.7 270 top
R31  85.5,57.4 0 top
R32  125.6,13.5 90 top
R33  136.4,15.75 270 top
R34  136.9,34.7 90 top
R35  107.6,30.9 0 top
R36  100.8,31.3 270 top
R37  109.9,27.5 0 top
R38  110.8,21.5 0 top
R39  91,21.6 180 top
R40  91.9,34.5 90 top
R41  81.1,33.3 0 top
R42  48,56.9 270 top
R43  48,79.2 90 top
R44  61,88 270 top
R45  45,102.8 0 top
R46  83.2,77.3 270 top
R47  45,100.4 0 top
R48  49.2,94.5 270 top
R49  83.2,86.3 90 top
R50  29,102.3 270 top
R51  68.3,90.6 0 top
R52  72.1,73.2 180 top
R53  86,69.7 0 top
R54  94.5,70.5 0 top
R55  94.5,68.1 180 top
R56  106.7,71.6 270 top
R57  85.6,77.3 90 top
R58  77.2,90.6 0 top
R59  94.5,88.3 0 top
R60  94.6,90.7 180 top
R61  106.7,86.1 90 top
R62  85.6,86.3 270 top
R63  92.2,102.6 270 top
R64  89.3,102.6 270 top
R65  102.2,102.2 180 top
R66  114.6,101.6 90 top
R67  114.4,88.4 0 top
R68  112.1,101.6 90 top
R69  112.3,70.6 0 top
R70  91.7,18.4 180 top
R71  113.1,18.2 180 top
R72  142.8,96.2 270 top
R73  142.8,84.8 270 top
R74  57.2,37.2 90 top
R75  54.8,37.2 270 top
S1  83.2,103.2 180 top
S2  54.4,103.2 180 top
T1  PN2222  [TO92-EBC']  46,4.7 90 top
TR1  29.4,45.2 90 top

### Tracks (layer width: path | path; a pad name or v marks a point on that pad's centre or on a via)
+14V
  Bottom 1: IC2.8 69.89,84.61 71.4,83.1 73.3,83.1 75,81.4 77,81.4 80,84.4 88.1,84.4 89.3,83.2 91.3,83.2 IC3.8 91.39,81.31 92.5,80.2 108.88,80.2 IC4.8 111.89,81.51 113.9,79.5 119.6,79.5 120.8,78.3 127.3,78.3 128.8,79.8 128.8,81.5 128.2,82.1 128.2,85 129.3,86.1 129.3,90.8 127.7,92.4 127.7,100.1 129,101.4 130.76,101.4 C56.2
  Bottom 1.2: Q18.E 144.96,91.96 143.6,90.6 138.9,90.6 136.7,92.8 133.11,92.8 C51.+ 131.5,94.41 C56.2
-14V  (via drill 0.8 pad 1.4)
  Top 0.8: v130.2,72.8 v135.4,72.8 | v140.4,76.8 v146.5,76.8
  Bottom 1: IC2.4 85.99,77.99 86,78 97.7,78 99,76.7 99,76.4 | 99,76.4 IC3.4 | 99,76.4 100.8,78.2 109.6,78.2 109.8,78 117.9,78 119.5,76.4 | 119.5,76.4 IC4.4 119.51,76.01 | 119.5,76.4 119.6,76.4 119.8,76.6 126.4,76.6 v130.2,72.8 | C52.- 133.1,84.06 C55.1 | v135.4,72.8 135.3,76.4
  Bottom 1.2: C52.- 133.45,76.65 133.81,76.4 135.3,76.4 139.6,76.4 v140.4,76.8 | v146.5,76.8 146.5,79.42 Q19.E
GND  (via drill 0.8 pad 1.5, 0.9 pad 1.5, 3.3 pad 6.6)
  Top 0.8: v67.9,8 v67.9,3.3
  Top 0.9: v6,50.5 v6,57 | v7.5,50.5 v7.5,57 | v9,50.5 v9,57 | v9,45 v9,38.5 | v7.5,45 v7.5,38.5 | v6,45 v6,38.5 | v6,33 v6,26.5 | v7.5,33 v7.5,26.5 | v9,33 v9,26.5 | v6,21 v6,14.5 | v7.5,21 v7.5,14.5 | v9,21 v9,14.5
  Bottom 1: CONN1.1 18.5,8 18.5,20.91 C2.- 17.8,23 18.7,23.9 18.7,30 20.4,31.7 42.6,31.7 44.2,33.3 45.2,33.3 46.69,33.3 R14.2 | v6,14.5 6,11.7 4.4,10.1 R20.2 4,9.79 v4,4 | T1.E 46.64,2.16 42.2,6.6 42.2,18.41 42.1,18.51 | R8.2 61.13,28.81 C8.2
  Bottom 1.2: v6,21 4.5,21 Q6.S | v6,21 v7.5,21 v9,21 | v9,14.5 9.1,14.4 9.1,7.4 CONN1.1 22.7,3.4 30.8,3.4 32.4,5 32.4,15.8 30.94,17.26 C1.1 34.34,17.9 C3.- 39.8,23.36 39.8,19.9 41.19,18.51 42.1,18.51 R2.1 44.4,18.34 C4.2 | v6,21 v6,26.5 | v6,33 v6,38.5 | v6,33 v7.5,33 v9,33 | v6,33 4.5,33 Q7.S | v6,45 4.5,45 Q4.S | v6,45 v7.5,45 v9,45 | v6,50.5 v6,45 | Q5.S 4.45,56.95 4.5,57 v6,57 v7.5,57 | v9,50.5 v7.5,50.5 | T1.E 49.9,2.16 | 49.9,2.16 54.63,2.16 R6.2 R9.2 64,1.99 | LED1.K 49.93,2.19 49.9,2.16 | 64,1.99 R10.2 67.61,3.3 v67.9,3.3 | C7.1 63.8,2.19 64,1.99 | IC1.7 68.85,8.95 v67.9,8 | 69.4,28.81 R12.2 62,28.81 | 69.4,28.81 R13.2 | 62,28.81 61.47,28.81 C8.2 | Q3.C 62.17,28.98 62,28.81 | Q2.C 69.37,28.84 69.4,28.81 | JP1.2 45.1,33.2 45.2,33.3 | C5.- 49.9,31.8 | 49.9,31.8 49.9,33.09 R15.2 R14.2 | R8.2 52.89,28.81 49.9,31.8
  Bottom 1.3: R21.2 3.69,57.71 4.45,56.95
  pour Bottom (isolate 0.6, rank 2, no thermals): 42.7,13.4 42.7,25 41.7,26 37.9,26 37.3,25.4 37.3,22.8 33.6,19.1 31.2,19.1 30.3,18.2 30.3,7.1 28.4,5.2 23.5,5.2 20.7,8 20.7,20.9 10.6,31 10.6,57.9 8.5,60 2.5,60 1.6,59.1 1.6,3.3 4.2,0.7 35.3,0.7 36.6,2 36.6,7.3
  pour Bottom (isolate 0.6, rank 3, no thermals): 35.5,1 36,1 36.5,0.5 74,0.5 76,2.5 76,34.5 71,39.5 60.5,39.5 59.5,38.5 48.5,38.5 44.5,42.5 44.5,48 41,51.5 36.5,51.5 33.5,48.5 24,48.5 23.5,48 23.5,33 22.5,32 22.5,31.5 23,31 34,31 37,28 40.5,28 41.5,27 41.5,14.5 34.5,7.5 34.5,2
GNDA  (via drill 0.8 pad 1.4, 0.8 pad 1.5)
  Top 0.8: v129.5,105.4 v129.5,99.3 | v45.3,85.5 v45.3,63.2 | v89.2,79.9 v89.2,74.8 | v109.8,75.1 v109.8,87.3 | v135.4,70.9 v126.8,70.9 | v112.7,68.4 v109.5,68.4 | v109.6,89.9 v126.1,89.9 | v73,70.3 v73,63.9
  Bottom 0.8: R42.2 54.45,47.9 59.7,47.9 64.3,43.3 72.5,43.3 80.65,35.15 | 80.9,34.9 80.9,22.8 | 80.9,22.8 80.9,17.6 80.9,6.3 85.1,2.1 | R43.2 50.95,85.55 52.6,87.2 56.6,87.2 59.3,84.5 59.3,83.5 64,78.8 65,78.8 66.6,77.2 66.6,72.5 67.8,71.3 71.7,71.3 v73,70.3 73.6,69.7 76.8,69.7 78.4,68.1 88.3,68.1 | 88.3,68.1 90,66.4 101.1,66.4 102.77,68.07 102.77,68.4 C39.- | v89.2,74.8 88.3,73.8 88.3,68.1 | C44.- 106.49,89.7 R61.2 | C21.- 80.82,22.88 80.9,22.8 | CON1.1 113.31,7.69 108.4,12.6 101.1,12.6 100.59,12.6 100.26,12.93 CON1.3 94.69,7.69 89.4,2.4 88.7,2.4 88.4,2.1
  Bottom 1: R62.2 R57.2 | C38.2 102.77,72.67 C39.- 102.8,68.87 | C43.2 102.64,89.47 C44.- | R63.1 110.6,106.41 R68.2 R66.2 122.9,105.41 | 122.9,105.41 129.11,105.41 v129.5,105.4 | 102.77,68.4 103.38,67.79 R56.2 106.7,68.81 R69.1 | R69.1 108.49,73.79 v109.8,75.1 | v109.8,87.3 109.8,87.61 | 109.8,87.61 R67.1 110.59,88.61 arc45 110.52,88.78 v109.6,89.9 | R61.2 109,87.61 109.8,87.61 | v135.4,70.9 136.5,70.9 140.1,74.5 140.6,74.5 142.1,76 142.1,77.7 140.5,79.3 D11.C | v126.8,70.9 125.9,70.9 124.7,69.8 121.5,69.8 120.1,68.4 v112.7,68.4 | v109.5,68.4 108.49,69.4 R69.1 | C55.2 132.8,89.59 arc45 132.73,89.77 129.6,92.9 129.6,99.09 arc45 129.53,99.27 v129.5,99.3 | v126.1,89.9 126.1,102.11 arc45 126.03,102.28 122.9,105.41 | C18.1 82.4,61.9 83.6,60.7 83.6,58.6 82.4,57.4 R31.1 | 80.9,34.9 79.8,34.9 | 79.8,34.9 79.59,34.9 R41.1 | C23.1 79.86,34.96 79.8,34.9
  Bottom 1.2: D10.A 138.09,97.1 C51.- 135.53,97.56 C53.- 133.09,105.74 C56.1 129.36,105.74 v129.5,105.4 | C55.2 132.7,89.3 136.2,85.8 136.67,85.8 C54.+ C52.+ 137.09,80.99 D11.C | C34.+ 26.77,100.72 R50.2 29,98.8 30.3,100.1 36.9,100.1 42.6,94.4 42.6,88.2 v45.3,85.5 | v45.3,63.2 31.65,60.6 31.05,66.9 | 48,57.9 R42.2 | 85.1,2.1 88.4,2.1 88.93,2.1 | C49.1 80.8,17.7 80.9,17.6 | R57.2 86.89,79.91 v89.2,79.9 | R64.1 R63.1
  Bottom 1.3: C29.1 C33.1 80.93,82.49 R49.1 | R46.1 R49.1 | R49.1 R62.2 | C50.1 101.66,13.16 101.1,12.6 | R31.1 80,57.4 77.76,59.64 C16.- 73,62.39 v73,63.9
  Bottom 1.4: 48,57.9 v45.3,63.2 | R43.2 45.35,85.55 v45.3,85.5
  Bottom 1.5: TR1.9 31.05,66.9 31.05,68.76 C13.+ | C24.+ C13.+ | C12.- 20.91,86.49 20.91,67.62 C25.- 28.2,66.11 C13.+
  pour Bottom (isolate 0.6, no thermals): 31.6,54.9 28.9,54.9 28.1,55.7 28.1,57.9 21.5,64.5 19.6,64.5 18.2,65.9 18.2,66.6 17.9,66.9 18.1,67.1 18.1,88.1 19.2,89.2 28.5,89.2 31,91.7 31.7,91.7 33.1,90.3 33.1,56.4
  pour Bottom (isolate 0.6, no thermals): 33.2,56.4 38.8,56.4 46.2,49 46.2,45.4 47.4,44.2 49,44.2 49.7,43.5 57.6,43.5 60.7,40.4 71.2,40.4 76.8,34.8 76.8,2.5 78.2,1.1 95.8,1.1 95.8,5.4 83.6,5.4 82.8,6.2 82.8,36.9 73.4,46.5 63.3,46.5 44.8,64.9 34.4,64.9 32.6,66.7 32.6,57
  pour Bottom (isolate 0.6, no thermals): 82.4,11.8 82.4,9.7 83.4,8.7 83.4,7.4 84.6,6.2 88,6.2 92.1,10.3 97.4,15.5 110.2,15.5 116.2,10.4 103.3,10.4 101.1,8.2 101.1,3.6 97.5,0.4 79,0.3 78.2,1.1 78.2,7.6
  pour Bottom (isolate 0.6, rank 2, no thermals): 106.4,10.8 105.6,10.8 110.1,6.4 110.3,6.2 116.2,6.2 116.7,6.7 116.7,9.9 116.1,10.5 107,10.5
  pour Bottom (isolate 0.6, rank 6, no thermals): 7.9,107.7 7.9,102.8 9.7,101 10,100.7 10.2,100.5 10.4,100.3 27.6,100.3 28.4,99.5 29.3,99.5 30.2,100.4 36.9,100.4 42.7,94.6 42.7,88.5 45.3,85.9 50.8,85.9 52.4,87.5 56.1,87.5 58.9,84.7 59,84.6 59,80.8 60.7,79.1 63.7,79.1 66.1,76.7 66.1,54.2 81.1,39.2 81.1,7.5 84.7,3.9 95.4,3.9 98.3,1 146.8,1 148.7,2.9 148.7,100.5 142,107.2 8.4,107.2
N$1
  Bottom 1: CONN1.2 25.86,9.04 C1.2 25.86,20.73 C2.+ 24.35,28.15 TR1.7 33.21,23.4 C3.+
  Bottom 1.2: IC1.8 71.39,13.21 66.3,18.3 IC1.11
  Bottom 1.4: 44.15,26.05 45.96,24.24 Q1.E 52.74,24.24 54.6,25.8 62.7,25.8 65.8,22.7 65.8,19.72 IC1.11 | 44.15,26.05 42.8,27.4 36.46,27.4 C3.+ | R4.2 45.5,27.4 44.15,26.05
  pour Bottom (isolate 0.6, no thermals): 28.3,5.4 23.5,5.4 20.9,8 20.9,21 19,22.9 19,30 19.9,30.9 36.1,30.9 37.1,29.9 37.1,23 33.4,19.3 31,19.3 30,18.3 30,7.1
N$2
  Bottom 1.2: C26.+ 59.68,93.13 R44.1
N$3
  Bottom 1.2: R1.2 42.91,1.89 CONN1.3
N$4
  Bottom 1: R1.1 44.4,7 46.7,4.7 T1.B
  Bottom 1.2: C4.1 44.57,11.06 R2.2 R1.1
N$5
  Bottom 1.2: R3.1 48.52,8.49 T1.C
N$6
  Bottom 1.2: Q1.B 48.4,19.16 | 48.4,19.16 46.63,19.16 R4.1 | R3.2 48.6,18.96 48.4,19.16
N$7  (via drill 0.8 pad 1.5)
  Top 0.8: v51.8,20.9 v51.8,26.7 | v54.3,15.8 v63.8,15.8
  Bottom 1.2: R5.1 51,16.2 51.8,17 | 51.8,17 v51.8,20.9 51,21.7 Q1.C | v54.3,15.8 53,15.8 51.8,17 | v63.8,15.8 63.8,19.18 IC1.12 | JP1.1 46.87,30.13 48.4,28.6 49.87,28.6 C5.+ 51.8,26.73 v51.8,26.7
N$8
  Bottom 1: R5.2 51,6.27 LED1.A
N$9
  Bottom 1.2: R74.1 57.31,33.39 58.7,32 58.7,31.34 OK1.1
N$10
  Bottom 1: IC1.3 58.71,11.59 58.8,11.5 58.8,7.7 57.1,6 C6.2
N$11
  Bottom 1: C6.1 57.1,9.9 56.2,10.8 56.2,11.54 IC1.2 IC1.15 56.15,21.66 R7.2
N$12  (via drill 0.8 pad 1.5)
  Top 1: v72,15.6 v66,15.6
  Bottom 1: R7.1 62.7,21.7 | 62.7,21.7 61.2,20.2 61.2,19.24 IC1.13 61.2,19.18 61.2,15.5 62.7,14 64.9,14 66,15.1 v66,15.6 | OK1.4 58.67,19.23 IC1.14 | C8.1 61.3,23.1 62.7,21.7 | C9.+ 71.1,8.3 74,11.2 R11.1 72.31,15.91 v72,15.6
  Bottom 1.2: IC1.14 IC1.13
N$13
  Bottom 1: IC1.16 R8.1 53.6,21.9 55.39,23.69 OK1.3
N$14
  Bottom 1.2: Q4.G 3.04,37.15 R16.1
N$15
  Bottom 1: R9.1 61.3,8.6 62.9,7 64.7,7 66.1,5.6 70.73,5.6 C9.- 71.13,5.2 71.9,5.2 74,7.3 R11.2
  Bottom 1.2: IC1.4 61.23,9.68 R9.1
N$16
  Bottom 1.2: IC1.5 63.77,9.67 C7.2
N$17
  Bottom 1.2: IC1.6 R10.1
N$18
  Bottom 1.2: Q5.G 3.04,49.15 R17.1
N$19
  Bottom 1: R20.1 11.7,10.1 13,11.5 13,14.1 13.9,15 15.69,15 C11.2
N$20  (via drill 0.8 pad 1.5)
  Top 0.8: v65.9,25.9 v65.9,31.1
  Bottom 1.2: IC1.10 68.85,19.84 R12.1 68,23.8 v65.9,25.9 64.81,26.99 D2.A | v65.9,31.1 64.3,31.1 62.8,32.6 Q3.B
N$21
  Bottom 1.2: IC1.9 71.39,20 R13.1 70.4,25.89 D1.A 72.3,30.4 70,32.7 Q2.B
N$22  (via drill 0.9 pad 1.5)
  Top 1: v11.3,38.4 v11.3,46.5 | v12.9,46.5 v42,46.5
  Bottom 1: v11.31,46.51 v11.3,46.5
  Bottom 1.2: v11.31,38.39 v11.3,38.4 | v42,46.5 42,44.3 43.5,42.8 48.2,42.8 49.7,41.3 R15.1 49.7,40 52,37.7 59.5,37.7 60.1,37.1 65,37.1 66.86,35.24 Q2.E 72.13,35.24 D1.C
  Bottom 1.3: R16.2 v11.31,38.39 | v11.3,46.5 v12.9,46.5 | R17.2 v11.31,46.51
N$23
  Bottom 1.2: Q6.G 3.04,13.15 R18.1
N$24  (via drill 0.9 pad 1.5)
  Top 0.9: v11,14.4 v11,22.5
  Top 1: v11.3,26.4 v11.3,34.5 | v13.4,40 v42,40
  Bottom 1: R18.2 11.31,14.4 v11,14.4 | v11.3,34.5 12.3,34.5 13.4,35.6 v13.4,40
  Bottom 1.2: D2.C 63.77,35.14 Q3.E 59.06,35.14 58.4,35.8 50.8,35.8 47.3,39.3 R14.1 42.91,40.91 v42,40
  Bottom 1.3: v11,22.5 11,23.9 R19.2 11.31,25.79 v11.3,26.4
N$25
  Bottom 1.2: Q7.G 3.04,25.15 R19.1
N$26
  Bottom 1: Q4.D 10,41 12.4,43.4 15.7,43.4 | 15.7,43.4 20.85,38.25 TR1.2 | Q5.D 12.3,53 12.6,53 16,49.6 16,43.7 15.7,43.4
  Bottom 1.2: C10.1 12.26,52.96 12.3,53
  pour Bottom (isolate 0.6, no thermals): 19,33.2 19,35.3 17.1,37.2 14.5,37.2 14.2,37.5 14.2,40.4 13.7,40.9 13,40.9 12.4,40.3 12.4,39.9 12.3,39.8 2.2,39.8 1.6,40.4 1.6,41.7 2.2,42.3 4.1,42.3 5.4,43.6 9.3,43.6 10.4,44.7 10.4,45.3 10.7,45.6 11.9,45.6 12,45.7 12.4,45.7 12.6,45.5 13.3,45.5 13.8,46 13.3,46 11.6,47.7 11.6,49.7 9.5,51.8 2.2,51.8 1.6,52.4 1.6,53.7 2.2,54.3 4,54.3 5.3,55.6 14.7,55.6 23.5,46.8 23.5,33.5 22.3,32.3 19.9,32.3
N$27
  Bottom 1: Q6.D 10.3,17 12.3,19 | 12.3,19 14,20.7 14,32.55 | Q7.D 10.45,29 14,32.55 | 14,32.55 TR1.1 | 12.6,18.7 C11.1 12.3,19
  pour Bottom (isolate 0.6, no thermals): 1.5,17.6 1.5,16.4 2.2,15.7 13.7,15.7 16,18 16,22.1 18.3,24.4 18.3,35 16.8,36.5 14.4,36.5 9.7,31.8 5.7,31.8 4.2,30.3 2.2,30.3 1.6,29.7 1.6,28.3 2.2,27.7 9.7,27.7 10.2,27.2 11.6,27.2 12.1,26.7 12.1,24.1 11.7,23.7 11.7,22.1 9.3,19.7 5.5,19.7 4.1,18.3 2.2,18.3
N$28
  Bottom 1.2: R21.1 11.01,58.93
  Bottom 1.3: 11.01,58.93 C10.2
N$29
  Bottom 1.2: IC1.1 53.61,10.8 R6.1
N$30
  Bottom 3: TR1.4 TR1.3
N$31
  Bottom 3: TR1.6 TR1.5
N$32
  Bottom 1: C27.+ 40.46,103.53 R45.1
N$33  (via drill 0.9 pad 1.5)
  Top 0.9: v8.1,75.4 v8.1,81.3 | v9.6,75.4 v9.6,81.3
  Bottom 1.5: D4.A2 4.64,79.54 6.95,81.85 | 6.95,81.85 8.9,83.8 8.9,87.3 7.2,89 D3.C | 6.95,81.85 7.8,81.3 v8.1,81.3 v9.6,81.3 | 11.7,70.6 9.6,72.7 v9.6,75.4 v8.1,75.4
  Bottom 2: TR1.10 25.85,56.4 23.4,56.4 12.3,68.2 11.7,70.6
  pour Bottom (isolate 0.6, rank 3, no thermals): 26.5,54.8 21.5,54.8 10,66.3 10,70.4 7.4,73 7.4,75.7 7.8,76.1 9.9,76.1 13.1,72.9 13.1,71.3 13.8,70.6 14.3,70.6 18.1,66.7 18.1,65.8 19.1,64.8 20,64.8 27.4,57.4 27.4,55.7
  pour Bottom (isolate 0.6, rank 3, no thermals): 2.2,78.8 5,78.8 6.9,80.6 9.9,80.6 10.3,81 10.3,88.3 8.5,90.3 2.2,90.3 1.6,89.7 1.6,88.4 2.2,87.8 6.4,87.8 7.4,86.8 7.4,84.5 6.6,83.7 1.7,83.7 1.5,83.5 1.5,79.5
N$34
  Bottom 1.5: D5.C 9.1,65 | 9.1,65 22.6,51.5 32.5,51.5 36.15,55.15 TR1.8 | D4.A1 4.54,74.46 8.9,70.1 8.9,65.2 9.1,65
  pour Bottom (isolate 0.6, rank 2, no thermals): 34.7,55.7 32.1,53.1 23,53.1 9.9,66.2 9.9,70.3 5,75.2 2.1,75.2 1.6,74.7 1.6,70.1 1.7,70 7,70 7.5,69.5 7.5,67.2 7,66.7 2.2,66.7 1.6,66.1 1.6,63.9 2.3,63.2 7,63.2 7.8,62.4 7.8,61.5 9.7,59.8 11.3,59.8 11.8,59.3 11.8,57.2 13,56 14.9,56 21.8,49.1 33.3,49.1 37.6,53.4 37.6,55.7
N$35
  Bottom 1: R22.2 144.67,44 Q9.S
  pour Bottom (isolate 0.6, no thermals): 139.1,43.6 139.1,44.8 141,46.7 146.4,46.7 147.4,45.7 147.4,43.7 146.4,42.7 140,42.7
N$36  (via drill 0.8 pad 1.4, 1.1 pad 1.7)
  Top 0.8: v96.8,42.1 v96.8,21.3 | v98.2,42.1 v98.2,21.3
  Top 1.1: v114.3,46.2 v114.3,56.3
  Bottom 0.8: R28.2 86.3,45.3 87.6,46.6 93,46.6 95.8,44 | 95.8,44 97.2,44 | 97.2,44 104.1,44 | 95.8,44 v96.8,42.1 | v96.8,21.3 96.8,20.75 R70.1 | v98.2,42.1 97.2,44
  Bottom 1: R22.1 114.28,44.28 v114.3,46.2 | C15.- 113.3,57.1 v114.3,56.3 114.19,58.22 R23.2
  Bottom 1.2: R70.1 87.34,7.69 CON1.4 | 114.3,45.6 112.8,44.1 104.2,44.1 104.1,44
  Bottom 1.7: v114.3,46.2 114.3,45.6
  pour Bottom (isolate 0.6, rank 2, no thermals): 94.4,45.9 105.2,45.9 105.5,46.2 114.8,46.2 115.1,45.9 115.1,43.6 112.4,40.7 97.2,40.7 94.4,43.5
  pour Bottom (isolate 0.6, rank 2, no thermals): 83.5,7.3 83.5,13.9 90,20.4 95,20.4 96.5,21.9 99.3,21.9 100.3,20.9 100.3,16.2 99.9,15.8 97.3,15.8 88.1,6.6 88,6.5 84.3,6.5
  pour Bottom (isolate 0.6, no thermals): 111,56.4 111,59 113.4,61.4 116,61.4 116.6,60.8 116.6,55.9 115.8,55.2 112.1,55.2
N$37
  Bottom 1: Q8.S 141.98,61.91 R23.1
  pour Bottom (isolate 0.6, rank 2, no thermals): 139.1,59.6 139.1,61.9 141,63.8 146.3,63.8 147.4,62.7 147.4,61.1 145.4,59.1 139.6,59.1
N$38
  Bottom 1.4: R27.2 128.95,50.95 130,49.9 134.1,49.9 136.4,52.2 D6.A 145.37,56.09 Q9.G
N$39
  Bottom 1.4: D6.C 133,52.2 137.7,56.9 140.78,56.9 D7.A
N$40  (via drill 0.8 pad 1.4)
  Top 0.8: v134.7,65.9 v129.9,65.9
  Bottom 1: Q8.G 145.57,73.1 144.3,73.1 140.8,69.6 | 140.8,69.6 138.3,67.1 135.9,67.1 v134.7,65.9 | D7.C 140.8,69.6 | C14.2 110.2,59.3 113.1,62.2 122.4,62.2 124.6,64.4 128.2,64.4 129.6,65.8 v129.9,65.9
  Bottom 1.2: Q10.C 100.6,58.26 C14.2
N$41
  Bottom 1.2: R24.1 103.2,55.5 Q10.E
N$42
  Bottom 0.8: R44.2 64.89,80.3 70.8,80.3 72.43,78.67 IC2.2
  Bottom 1.2: IC2.2 72.43,76.31 C36.1 C28.2 74.66,74.45 R52.1
N$43
  Bottom 0.8: R26.2 111.35,52.7 107.4,52.7 106.6,53.5 106.6,55.8 107.9,57.1 C15.+
  Bottom 1: R26.2 115.6,52.65 R27.1
N$44
  Bottom 1.2: Q10.B 98.06,57.8 C14.1
  Bottom 1.3: Q12.C 96.9,54.67 | 96.9,54.67 97.17,54.67 Q10.B | R25.1 97,54.57 96.9,54.67
N$45
  Bottom 1.3: R28.1 85.3,53.41 Q11.B 85.3,56.5 88.5,59.7 R29.1
N$46
  Bottom 0.8: R45.2 46.3,100.3 46.3,88.9 47.9,87.3 50.6,87.3 51.9,88.6 57.2,88.6 58.7,87.1 60.8,87.1 66.3,81.6 72.1,81.6 75,78.7 75,78.02 IC2.3 75.1,77.86 75.1,77.3 77,75.4 C28.1 | R46.2 83.2,73.76 C29.2
  Bottom 1.2: C29.2 80.24,75.4 C28.1
N$47
  Bottom 1.2: R30.1 89.3,53.9 | 89.3,53.9 89.3,54.63 Q12.E | Q11.E 89.13,53.73 89.3,53.9
N$48
  Bottom 1.3: R29.2 80.71,59.7 C16.+
N$49
  Bottom 1.2: R31.2 92,57.4 | 92,57.4 92.47,57.4 C17.+ | Q12.B 91.8,57.2 92,57.4
N$50  (via drill 0.8 pad 1.5)
  Top 1: v58.2,97.7 v51.9,97.7
  Bottom 1: v58.2,97.7 61.8,97.7 62.7,96.8 64.1,96.8 65,97.7 71.34,97.7 CONN2.T1 | v51.9,97.7 51.9,100.62 S2.3
N$51  (via drill 1.1 pad 1.8)
  Top 1.1: v142.4,11 v142.4,20.4
  Bottom 0.8: Q14.S 142.89,10.91 v142.4,11 | R32.2 128.84,27.57 134.7,21.7 141.1,21.7 v142.4,20.4
  pour Bottom (isolate 0.6, no thermals): 141.9,13 147,13 147.4,12.6 147.4,8.4 147.1,8.1 141.8,8.1 141.2,8.7 141.2,12.3
  pour Bottom (isolate 0.6, rank 2, no thermals): 124.7,27.9 124.7,26.4 132.2,18.9 142.7,18.9 143.2,19.4 143.2,22.3 143,22.5 137,22.5 131,28.5 129.3,28.5 129.2,28.6 125.4,28.6
N$52
  Bottom 0.8: 125.6,2.29 126.2,1.69 | CON1.2 104.62,7.48 110.3,1.8 119.1,1.8 | 119.1,1.8 125.49,1.8 R32.1 | 119.45,2.15 119.1,1.8
  Bottom 1: C20.- 104.23,18.63 105.5,19.9 113.01,19.9 R38.2
  Bottom 1.4: R33.2 126.2,1.69 R32.1 | 119.45,2.15 118.9,2.7 118.9,4.2 119.45,4.75 R71.1 117.91,18.2 R38.2
  pour Bottom (isolate 0.6, no thermals): 102.7,8 102.7,1.8 103.9,0.6 137.1,0.6 138,1.5 138,4.7 136.4,6.3 115.9,6.3 115.3,5.7 109.2,5.7 106.4,8.5 103.2,8.5
N$53
  Bottom 1.8: R33.1 136.53,27.57 139.1,25 142.67,25 Q13.S
  pour Bottom (isolate 0.6, no thermals): 135.8,28.5 141.1,28.5 143.2,30.6 147,30.6 147.5,30.1 147.5,24.8 146.9,24.2 144.4,24.2 143.4,23.2 135.9,23.2 135.2,23.9 135.2,27.9
N$54  (via drill 0.8 pad 1.4)
  Top 0.8: v123.4,27.5 v120.4,27.5
  Bottom 0.8: Q14.G 145.58,20.88 143.1,18.4 131.9,18.4 123.4,26.9 v123.4,27.5
  Bottom 1.3: D8.A 111.5,24 115,27.5 R37.2 v120.4,27.5
N$55
  Bottom 0.8: D9.A 141.9,29.3 140.6,28 138.9,28 137.5,29.4 122.8,29.4 121.9,28.5 121.9,26.1 119.8,24 D8.C
N$56  (via drill 0.8 pad 1.4)
  Top 0.8: v139.7,40.8 v139.7,29.6
  Bottom 0.8: v139.7,29.6 139.7,30.8 136.1,34.4 131,34.4 130.5,33.9
  Bottom 1.2: 139.72,40.78 v139.7,40.8
  Bottom 1.3: Q15.C 130.5,33.9 130.5,35.06 C19.2
  Bottom 1.4: Q13.G 143.89,40.78 D9.C 139.72,40.78
N$57
  Bottom 1.3: R34.1 135.83,31.96 Q15.E
N$58
  Bottom 1.2: C34.- 27.17,104.28 R50.1 32.96,106.11 C30.- C27.- 48.23,106.07 51.2,103.1 64.69,103.1 CONN2.S
N$59  (via drill 0.8 pad 1.4)
  Top 0.8: v90.7,25.6 v94.9,25.6
  Bottom 1: R35.1 103.79,30.71 105.3,29.2 119.8,29.2 122.5,31.9 127.9,31.9 Q15.B
  Bottom 1.2: v94.9,25.6 98.49,25.6 R35.1
  Bottom 1.3: v90.7,25.6 86.8,25.6 84.3,28.1 84.3,29.19 Q17.C
  Bottom 1.4: Q15.B 127.96,33.4 C19.1
N$60
  Bottom 1.1: C20.+ 101.5,24.25 R36.2
  Bottom 1.3: R37.1 103.35,27.5 R36.2
N$61
  Bottom 1: C30.+ 34.57,103.53 36.4,101.7 39.89,101.7 R47.1
N$62  (via drill 0.8 pad 1.4)
  Top 0.8: v99.7,23.2 v103.3,23.2
  Bottom 1.2: R38.1 104.4,21.5 103.3,22.6 v103.3,23.2
  Bottom 1.3: Q16.B 92.7,23.71 94.46,21.95 | 94.46,21.95 R39.1 | v99.7,23.2 95.7,23.2 94.46,21.95
N$63
  Bottom 1.3: Q16.E 90.16,28.95 | 90.16,28.95 R40.1 | Q17.E 89.88,29.23 90.16,28.95
N$64
  Bottom 1.4: R39.2 85.78,21.6 C21.+
N$65
  Bottom 1.3: Q17.B 86.8,31.41 86.71,31.5 | 86.71,31.5 R41.2 | C22.+ 88.1,32.9 86.71,31.5
N$66
  Bottom 1.2: C49.2 84.65,17.7 R70.2
N$67
  Bottom 0.8: C31.+ 53.07,93.1 52.8,93.1 49.2,96.7 R48.1
N$68  (via drill 0.8 pad 1.4)
  Top 0.8: v68,83.3 v76.2,83.3
  Bottom 0.8: R47.2 48.81,100.31 47.6,99.1 47.6,89.8 48.7,88.7 49.7,88.7 51,90 57.9,90 59.2,88.7 62.59,88.7 R51.1 | v76.2,83.3 76.1,83.3 75,84.4 75,85.58 IC2.6 | v68,83.3 68,87.56 C35.1
  Bottom 1: C35.1 67.19,88.2 R51.1
  Bottom 1.3: IC2.6 74.97,87.49 C32.2
N$69  (via drill 0.8 pad 1.4)
  Top 0.8: v66.5,92.4 v79.5,92.4
  Bottom 0.8: C33.2 80.4,87.54 C32.1 79.4,88.54 79.4,92.3 v79.5,92.4 | v66.5,92.4 64,92.4 61.8,90.2 60,90.2 58.8,91.4 50.3,91.4 49.59,90.69 R48.2
  Bottom 1: C33.2 83.2,89.84 R49.2
  Bottom 1.3: IC2.5 77.51,86.37 C32.1
N$70
  Bottom 0.8: R51.2 72.11,88.53 C35.2
  Bottom 1: IC2.7 C35.2 | R51.2 R58.1 78.39,95.6 C46.+
N$71  (via drill 0.8 pad 1.5)
  Top 1: v61.6,100.7 v61.6,95.3
  Bottom 1: S2.1 61.16,100.66 v61.6,100.7 | C26.- 60.93,95.67 v61.6,95.3 65.89,95.3 CONN2.T2
N$72
  Bottom 1: S2.2 54.4,96.97 C31.-
N$73
  Bottom 1: R53.2 89.89,69.7 R54.1 90.66,70.53 C37.1
N$74
  Bottom 1: R52.2 73,73.2 74.8,71.4 78.23,71.4 C41.+ 78.5,71.67 78.5,71.1 79.9,69.7 R53.1
  Bottom 1.2: R52.2 68.26,73.23 C36.2 68.26,76.36 IC2.1
N$75
  Bottom 1: IC3.3 96.4,75.42 96.4,74.9 97.56,73.74 C38.1 98.31,72.05 R54.2
N$76
  Bottom 1: IC3.1 IC3.2 93.93,74.61 C37.2 95.7,72.76 95.7,71.7 92.1,68.1 R55.2
N$77
  Bottom 1: R55.1 99.43,68.1 C39.+ 100.23,73.03 102,74.8 102,76.07 C40.+
N$78  (via drill 0.8 pad 1.4)
  Top 0.8: v108.1,91.2 v108.1,76.4
  Bottom 0.8: S1.1 86,100.3 86,96.2 87.7,94.5 88.8,94.5 90.9,92.4 99,92.4 100,91.4 107.4,91.4 v108.1,91.2
  Bottom 1: v108.1,76.4 106.6,76.4 | 106.6,76.4 104.87,76.4 C40.- | R56.1 106.7,76.3 106.6,76.4
N$79  (via drill 0.8 pad 1.4)
  Top 0.8: v87.4,86.2 v87.4,75.9
  Bottom 0.8: S1.3 80.7,100.62 80.7,99.2 85.4,94.5 85.4,92.8 87.4,90.8 v87.4,86.2 | R57.1 83.51,71.7 C41.-
  Bottom 1: R57.1 85.61,74.11 v87.4,75.9
N$80  (via drill 0.8 pad 1.4)
  Top 0.8: v90.8,100.2 v90.8,104.5 | v120,91.3 v120,102.4
  Bottom 0.7: v120,102.4 120,102.5 119.1,103.4 110.7,103.4 109,105.1 93.5,105.1 92.9,104.5 v90.8,104.5
  Bottom 0.8: S1.5 83.2,104.6 84.5,103.3 87.19,103.3 90.29,100.2 v90.8,100.2 91.09,99.9 R63.2 | IC4.5 119.51,83.91 arc-45 119.58,84.08 120.9,85.4 120.9,90.4 v120,91.3
N$81  (via drill 0.8 pad 1.4)
  Top 0.8: v82.2,92.7 v88,92.7
  Bottom 0.8: R58.2 81.01,91.51 v82.2,92.7 | R59.1 89.7,88.3 88.7,89.3 88.7,92 v88,92.7
  Bottom 1.3: R59.1 90.66,88.27 C42.1
N$82
  Bottom 1: IC3.5 99.01,84.35 C43.1 98.31,86.55 R59.2
N$83
  Bottom 1.3: IC3.7 95.7,83.11 | 95.7,83.11 IC3.6 | 95.7,83.11 95.7,85.76 C42.2 95.74,86.26 91.3,90.7 R60.2
N$84
  Bottom 0.8: C44.+ 99.21,89.7 R60.1
  Bottom 1: C44.+ 100.33,85.47 101.9,83.9 101.9,82.37 C45.+
N$85
  Bottom 0.8: S1.4 87.16,105.74 90.6,102.3 93.2,102.3 94.6,100.9 94.6,94.8 95.5,93.9 99.7,93.9 100.9,92.7 109.1,92.7 112.3,89.5 112.3,87 110.7,85.4 109.81,85.4 R61.1
  Bottom 1: R61.1 C45.-
N$86
  Bottom 0.8: S1.6 78.8,103.88 78.8,98.9 81.37,96.33 C46.- 81.4,95.47 81.6,95.7 83.9,93.4 83.9,92 85.6,90.2 R62.1
N$87  (via drill 0.8 pad 1.4)
  Top 0.8: v84.3,97.9 v87.7,97.9 | v91.5,94.1 v114.7,94.1 | v121.5,82.6 v121.5,75
  Bottom 0.7: IC4.3 117,75.56 117,74.8 118.5,73.3 120.3,73.3 121.5,74.5 v121.5,75 | v114.7,94.1 116.3,94.1 117.2,93.2 120.7,93.2 122.1,91.8 122.1,84.5 121.5,83.9 v121.5,82.6
  Bottom 0.8: S1.2 83.2,99.2 v84.3,97.9 | v91.5,94.1 89.6,96 88.5,96 87.7,96.8 v87.7,97.9 88.59,98.79 R64.2
N$88  (via drill 0.8 pad 1.4)
  Top 0.8: v125.3,82.6 v125.3,75 | v123.7,71.7 v118.3,71.7
  Bottom 0.7: v125.3,82.6 125.3,83.7 124.5,84.5 124.5,93.5 118.8,99.2 118.8,101.3 117.8,102.3 110,102.3 108.3,104 104,104 R65.1-2
  Bottom 0.8: v125.3,75 125.3,73.5 v123.7,71.7 | v118.3,71.7 117.34,71.7 C47.1
  Bottom 1: IC4.2 114.43,74.61 C47.1
N$89  (via drill 0.8 pad 1.4)
  Top 0.8: v123.4,82.6 v123.4,75
  Bottom 0.7: v123.4,82.6 123.3,82.8 123.3,92.6 114.7,101.2 108.4,101.2 107.4,102.2 R65.1-1 | C18.2 86.9,61.9 87.5,61.3 91.97,61.3 C17.-
  Bottom 0.8: v123.4,75 123.4,74.3 119.2,70.1 116.7,70.1 116.2,70.6 R69.2 | C17.- 92.9,60.7 93.4,61.2 105.1,61.2 106.1,62.2 109.8,62.2 111.1,63.5 111.1,69.8 112.63,71.33
  Bottom 1.2: R69.2 113.36,70.6 112.63,71.33 C47.2
  Bottom 1.3: IC4.1 111.89,73.73 C47.2
N$90
  Bottom 0.7: R66.1 112.24,100.15 99.25,100.15 R65.1-3
N$91
  Bottom 1: OK1.2 54.8,32.64 R75.2 54.7,33.29 D13.C
N$92  (via drill 0.8 pad 1.5)
  Top 0.8: v112.7,91.4 v116.8,91.4
  Bottom 0.7: R65.2-2 105,94 109.7,94 112.3,91.4 v112.7,91.4 | C48.1 119.7,87.16 119.7,89 117.4,91.4 v116.8,91.4
  Bottom 1: IC4.6 116.97,84.13 C48.1
N$93  (via drill 0.8 pad 1.4)
  Top 0.8: v127.1,80.6 v127.1,73.3 | v108.2,54.4 v108.2,39.9 | v93.7,43.3 v93.7,32.2
  Bottom 0.7: R65.2-1 108.5,95.9 110.6,95.9 115.2,91.3 115.2,90.2 116.16,89.24 116.16,88.4
  Bottom 0.8: IC4.7 114.43,82.17 115.6,81 121.2,81 122.13,80.07 arc45 122.31,80 126.4,80 arc45 126.57,80.07 v127.1,80.6 | v108.2,54.4 116.7,54.4 125,62.7 129.9,62.7 131.6,64.4 131.6,67 128.7,69.9 128.7,71.5 127.1,73.1 v127.1,73.3 | v108.2,39.9 96.6,39.9 93.7,42.8 v93.7,43.3
  Bottom 1: IC4.7 114.43,85.13 C48.2 116.16,88.4 R67.2 | C23.2 88.33,35.7 C22.- 88.47,35.7 89.4,35.7 92.9,32.2 v93.7,32.2
N$94
  Bottom 0.7: R65.2-3 99.1,99.1 111.2,99.1 112.1,98.2 R68.1
N$95
  Bottom 1.3: R71.2 C50.2
N$96  (via drill 3.3 pad 6.6)
  other vias: 4,104
N$97  (via drill 3.3 pad 6.6)
  other vias: 145,4
N$98  (via drill 3.3 pad 6.6)
  other vias: 145,104
N$99  (via drill 0.8 pad 1.4, 0.9 pad 1.5)
  Top 0.8: v117.7,38.3 v117.7,22.2 | v119.1,22.2 v119.1,38.3
  Top 0.9: v68,62.1 v68,53.5 | v69.5,62.1 v69.5,53.5
  Bottom 0.8: 113.25,37.55 111.4,39.4 | Q9.D 144.98,49.9 140.4,49.9 134.2,43.7 121.4,43.7 119.2,41.5 | v117.7,22.2 v119.1,22.2 120.2,21 124.8,16.3 145.68,16.3 Q14.D | v117.7,38.3 114,38.3 113.7,38
  Bottom 0.9: F1.1A 55.49,63.29 58.1,65.9 66.9,65.9 68,64.8 v68,62.1 v69.5,62.1 | v69.5,53.5 v68,53.5
  Bottom 1: v69.5,53.5 73.9,50.7 82.2,42.4 86.9,42.4 89.3,44.8 | 89.3,44.8 R30.2 | R26.1 111.4,39.4 111.4,39 109.5,37.1 97,37.1 95.15,38.95 | 95.15,38.95 89.3,44.8 | R40.2 94.51,38.31 95.15,38.95
  Bottom 1.2: R36.1 113.7,38 113.25,37.55
  Bottom 1.4: v117.7,38.3 v119.1,38.3 119.2,41.5
  pour Bottom (isolate 0.6, rank 3, no thermals): 67.3,50.4 67.3,53.5 68,54.2 74.3,54.2 82.6,45.9 92.9,45.9 94.2,44.6 94.2,43.4 97.1,40.5 112.4,40.5 115.5,43.8 115.5,45.6 115.9,46 120.8,46 126.6,51.8 142.3,51.8 143.1,52.6 146.5,52.6 147.4,51.7 147.4,48.7 145.7,47 140.9,47 135.3,41.4 122.8,41.4 115.1,33.7 93.1,33.7 89.7,37.1 83.4,37.1 71.7,48.8 68.9,48.8
  pour Bottom (isolate 0.6, rank 2, no thermals): 117,20.2 117,22.6 117.6,23.2 126.2,23.2 131.5,17.9 144,17.9 144.5,18.4 147.1,18.4 147.4,18.1 147.4,14.3 144.6,12 127.1,12 119.4,19.7 117.5,19.7
  pour Bottom (isolate 0.6, rank 3, no thermals): 53.9,62.3 52.4,63.8 52.4,66 53.5,67.1 53.5,67.9 53.5,68.9 54.4,69.8 55.6,69.8 56.5,68.9 60,68.9 61.1,67.8 64.1,67.8 65.1,68.8 69.1,68.8 70.6,67.3 70.6,65.2 71.3,64.5 71.3,64.1 71.3,62.7 69.9,61.3 66.6,61.3 64.8,63.1 60.8,63.1 59.5,61.8 54.4,61.8
N$101
  Bottom 1.2: Q18.B 145.57,97.04 R72.1 142.59,100 142,100 140.3,101.7 D10.C 138.86,102.51 C53.+
N$102
  Bottom 1.2: Q19.B 142.8,88.2 R73.1 D11.A 140.26,88.37 C54.-
N$104  (via drill 0.8 pad 1.4)
  Top 0.8: v105.1,47.2 v105.1,32.8 | v106.5,32.8 v106.5,47.2
  Bottom 0.8: v105.1,32.8 106,32.8 v106.5,32.8 107.5,31.8 118,33.4 122.5,37.1 137.5,37.1 141.1,33.5 Q13.D | v105.1,47.2 103.2,47.4
  Bottom 1: 103,49.9 118.4,49.9 125.9,57.4 131.9,57.4 140.2,65.7 143.2,65.7 145,67.5 Q8.D | 103,49.9 96.7,49.9 | 96.7,49.9 82.4,49.9 82.1,50.2 | 82.1,50.2 75.3,57 64.21,57 F2.1A | Q11.C 82.76,50.86 82.1,50.2 | R25.2 97,49.6 96.7,49.9 | R24.2 103.2,47.4 103.2,49.7 103,49.9 | Q16.C 95.24,30.84 97.2,32.8 v105.1,32.8
  Bottom 1.2: 105.91,32.71 106,32.8
  pour Bottom (isolate 0.6, no thermals): 144.8,69.3 142.8,67.3 139.6,67.3 138.7,66.4 136.6,66.4 130.7,60.5 124.9,60.5 116.3,51.9 116.3,52.5 84.9,52.5 77.5,59.2 67.2,59.2 64.1,62.3 60.8,62.3 58.8,60.3 58.8,55.5 60.8,53.5 66,53.5 67.4,54.9 74,54.9 82.2,46.6 120.6,46.5 129.9,55.4 132.3,55.4 140.9,64 144.7,64 147.4,66.7 147.4,68.2 146.3,69.3
  pour Bottom (isolate 0.6, no thermals): 105.2,33.9 114.8,33.9 122,41.1 141.2,41.1 144.3,35.4 146.3,35.4 147.4,34.3 147.4,32.7 146.2,31.5 139.2,31.5 136.4,34.3 123.1,34.3 119,30.2 105.1,30.2 104.3,31 104.3,32.8
VDD  (via drill 0.8 pad 1.4, 0.8 pad 1.5, 2.3 pad 4.5)
  Top 0.8: v49.5,64.9 v49.5,72.9 | v133.3,67.4 v128.3,67.4 | v112.7,64.4 v109.5,64.4 | v71.4,65.9 v71.4,47.9 | v127.6,88.3 v127.6,103.5 | v127.6,87.1 v131.1,87.1
  Top 1: v52.7,44.1 v52.7,59
  Top 2: v15.2,79.8 v42.7,79.8
  Bottom 0.8: v49.5,72.9 48.15,72.9 R43.1 | F1.2A 53.01,84.71 45.4,77.1
  Bottom 1: R75.1 54.8,42 v52.7,44.1 | v49.5,64.9 49.5,64.61 arc45 49.57,64.43 52.9,61.1 52.9,59.11 arc-45 52.83,58.93 v52.7,59 | v127.6,87.1 v127.6,88.3 | v127.6,103.5 131.59,103.5 arc-45 131.77,103.43 133.4,101.8 133.4,96 arc45 133.47,95.83 134.7,94.6 137.4,94.6 arc-45 137.57,94.53 139.4,92.7 142.38,92.7 arc-45 142.56,92.63 R72.2
  Bottom 1.2: R74.2 R75.1 | Q18.C 144.4,94.5 142.8,92.9 R72.2 | v131.1,87.1 131.1,85.2 130.8,84.9 130.8,79 130.2,78.4 130.2,76 133.23,72.97 arc-45 133.3,72.8 v133.3,67.4 | v128.3,67.4 127.2,66.3 124,66.3 arc45 123.83,66.23 122,64.4 v112.7,64.4 | v109.5,64.4 108.9,64 104.91,64 arc45 104.73,63.93 103.7,62.9 88.41,62.9 arc-45 88.33,62.97 86.7,64.6 76.3,64.6 75.07,65.83 arc45 74.9,65.9 v71.4,65.9 | v71.4,47.9 64,47.9 arc-45 63.63,48.17 v52.7,59
  Bottom 1.4: R43.1 48,74.5 45.4,77.1 v42.7,79.8
  Bottom 1.5: D4.C 5.5,77 6.3,77.5 10.91,77.5 14.41,74 C25.+
  Bottom 2: C25.+ 14.92,79.52 v15.2,79.8 14.41,80.59 C12.+
  pour Bottom (isolate 0.6, rank 5, no thermals): 1.5,77.8 1.5,76.2 2.2,75.5 6.9,75.5 7.7,76.3 10.2,76.3 13.4,73.1 13.4,72.2 14.8,70.8 16.9,70.8 17.4,71.3 17.4,92.7 15.2,94.7 12.8,94.7 10.5,92.5 10.5,80.7 10,80.2 6.6,80.1 5,78.5 2.2,78.5
  pour Bottom (isolate 0.6, no thermals): 41.9,81.8 41.9,83.9 42.9,84.9 47.7,84.9 49.2,86.4 57.6,86.4 58.7,85.3 58.7,81.1 49.8,72.2 42.5,72.2 41.9,72.8
VSS  (via drill 0.8 pad 1.4, 0.8 pad 1.5, 0.9 pad 1.5)
  Top 0.8: v135.3,69 v126.8,69 | v112.7,66.4 v109.5,66.4
  Top 0.9: v5.1,86.4 v5.1,91.6 | v6.6,91.6 v6.6,86.4 | v6.6,84.9 v6.6,69.1 | v5.1,69.1 v5.1,84.9 | v5.1,67.6 v5.1,61.8 | v6.6,61.8 v6.6,67.6
  Top 1: v50.7,43.3 v50.7,60.3
  Bottom 0.8: F2.2A 59.7,76.41 57.01,76.41 50.3,69.7 39.71,69.7 C13.-
  Bottom 1: 37.1,88.19 37.1,91.6 32.1,96.6 11.7,96.6 6.7,91.6 v6.6,91.6 | D13.A 52.2,41.8 v50.7,43.3 | v50.7,60.3 48,63 R42.1 45.15,66.1 41.4,66.1 39.21,68.29 C13.- | R73.2 142.8,79.61 arc45 142.87,79.43 143.9,78.4 143.9,75.7 arc-45 143.83,75.53 137.3,69 v135.3,69 | v126.8,69 126.91,69 arc45 126.73,68.93 125.9,68.1 122.91,68.1 arc45 122.73,68.03 121.17,66.47 arc-45 121,66.4 v112.7,66.4 | v109.5,66.4 108.71,66.4 arc45 108.53,66.33 108.1,65.9 103.41,65.9 arc45 103.23,65.83 102.2,64.8 89.41,64.8 arc-45 89.13,64.87 87.7,66.3 77.5,66.3 arc-45 77.23,66.47 75.7,68 72.31,68 arc-45 72.13,68.07 70.6,69.6 64.81,69.6 arc45 64.73,69.53 64.1,68.9 61.6,68.9 arc-45 61.43,68.97 59.7,70.7 59.7,76.41
  Bottom 1.2: Q19.C 144.31,82.5 R73.2
  Bottom 1.5: v5.1,67.6 v5.1,69.1 v6.6,69.1 v6.6,67.6 v5.1,67.6 | v5.1,86.4 v5.1,84.9 v6.6,84.9 v6.6,86.4 v5.1,86.4 | D3.A2 3.1,91.6 v5.1,91.6 v6.6,91.6 | v5.1,67.6 3.1,67.6 D5.A2 | v5.1,86.4 3.1,86.4 D3.A1 | v6.6,61.8 v5.1,61.8 3.7,61.8 D5.A1
  Bottom 2: C13.- 38.8,69.2 37.1,70.9 37.1,88.19 C24.-
  pour Bottom (isolate 0.6, rank 4, no thermals): 6.8,84.2 1.7,84.2 1.5,84.4 1.5,86.4 2.2,87.1 3.9,87.1
  pour Bottom (isolate 0.6, rank 4, no thermals): 6.6,66.9 2.1,66.9 1.6,67.4 1.6,69.5 1.7,69.6 4.6,69.6 5,69.2 5,68.5
  pour Bottom (isolate 0.6, rank 6, no thermals): 39.8,67.6 34.9,67.6 33.3,69.2 33.3,91 32.3,92 31,92 28.4,89.4 17.6,89.4 17.6,92.8 15.4,95 12.7,95 10.4,92.7 10.4,91.6 9.5,90.7 1.9,90.7 1.5,91.1 1.5,94.4 3.4,96.3 6.9,96.3 10.2,99.6 35.2,99.6 41.2,93.6 41.2,82.8 39.8,81.4 39.8,78.1 41.2,76.7 41.2,69
  pour Bottom (isolate 0.6, rank 2, no thermals): 41.2,74 41.2,72.6 42.3,71.5 49.7,71.5 56.9,78.7 65.1,78.7 66.5,77.3 66.5,70.6 65.4,69.5 56.7,69.5 55.7,70.5 50.9,65.6 49,65.6 47.7,64.1 45.6,65 45,65.6 35.1,65.6 33.9,66.8 33.9,71.6 36.5,75.1

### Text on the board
Bottom: 05/07/15 | V1 | ACP | ©
tPlace: PUSH / BRIDGE | IN | VOLUME | LPF | - | + | OUT | _ | _ | + | + | BRIDGE | _ | GND | REM | V+ | +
